(* Logix 5000 AddOnInstructionDefinition export Banner_K50Select_Param_v4; software revision 33.03 *)

TYPE Banner_IOL_Port_v4 :   // UDT that has all of the data items necessary to communicate with a specific Port on a IO-Link Master
STRUCT
   Port_Controlled : INT;   // Each bit represents a port on an IO-Link Master. Set to 1 to tell AOI to control that port.
   Port_Activate : INT;   // Each bit represents a port on an IO-Link Master. When ON that port will process any commands in queue.
   Port_Read : INT;   // Each bit represents a port on an IO-Link Master. Used to determine when device AOI has requested a Read command.
   Port_Write : INT;   // Each bit represents a port on an IO-Link Master. Used to determine when device AOI has requested a Write command.
   Port_RW_Complete : INT;   // Each bit represents a port on an IO-Link Master. Tells device AOI that Read or Write request has been completed.
   Port_Device_Read : INT;
   Data_Transfer : SINT[190];   // Array to transfer data from IO-Master to device AOIs.
END_STRUCT
END_TYPE

TYPE Banner_K50Select_DeviceLocks_v4 :
STRUCT
   Parameter_Access_Lock : SINT;   // Write access to all read/write parameters is block when this bit is ON.
   Data_Storage_Lock : SINT;   // Data storage mechanism is inhibited when bit is ON.
   Local_Parameterization_Lock : SINT;   // Parameteriation via local control elementes is inhibited.
   Local_User_Interface_Lock : SINT;   // Operation of the hmi on the device is disabled.
END_STRUCT
END_TYPE

TYPE Banner_K50Select_Direct_v4 :
STRUCT
   Master_Cycle_Time : INT;
   Min_Cycle_Time : INT;
   M_Sequence_Capability : INT;
   IO_Link_Version_ID : INT;
   Process_Data_Input_Length : INT;
   Process_Data_Output_Length : INT;
   Combined_Vendor_ID : DINT;   // IO-Link Vendor ID
   Vendor_ID1 : INT;
   Vendor_ID2 : INT;
   Combined_Device_ID : DINT;   // IO-Link Device ID
   Device_ID1 : INT;
   Device_ID2 : INT;
   Device_ID3 : INT;
END_STRUCT
END_TYPE

TYPE Banner_K50Select_InputSettings_v4 :
STRUCT
   Touch_Sensitivity : SINT;   // K50 Select touch models only. 0 = Low, 1 = High.
   Function : SINT;   // 0 = Momentary, 1 = Latched.
   Mute_Enable : SINT;   // 0 = Off, 1 = On.
   On_Delay : DINT;   // 0 to 65535 in ms. Length of time the touch button needs to be pressed to trigger touch active state.
   Target_Threshold_Low : DINT;   // K50 Select Sensor Models Only. 0 to 1500 Range in mm.
   Targer_Threshold_High : DINT;   // K50 Select Sensor Models Only. 0 to 1500 Range in mm.
   Min_Distance : DINT;   // K50 Select Sensor Models Only. 0 to 1500 Range in mm.
   Max_Distance : DINT;   // K50 Select Sensor Models Only. 0 to 1500 Range in mm.
END_STRUCT
END_TYPE

TYPE Banner_K50Select_Output_Settings_v4 :
STRUCT
   Output_State : SINT;   // 0 = NO, 1 = NC.
   Off_Delay_Type : SINT;   // 0 = Leading Edge, 1 = Trailing Edge.
   Off_Delay : DINT;   // 0 to 65535 in ms. Length of time before the device returns to the 'touch inactive' state after button is released.
END_STRUCT
END_TYPE

TYPE Banner_K50Select_RD_v4 :   // UDT with all of the Read only parameters for K50 Pro Select.
STRUCT
   Direct_Parameters : Banner_K50Select_Direct_v4;
   Serial_Number : STRING;
END_STRUCT
END_TYPE

TYPE Banner_K50Select_Settings_v4 :
STRUCT
   Custom_Intensity : SINT;   // 0 to 100 %
   Custom_Flash_Rate : INT;   // Range 5 to 200 (.5 to 20 converted rate).
   Restrict_to_Gamut : SINT;   // 0 = Off, 1 = On.
END_STRUCT
END_TYPE

TYPE Banner_K50Select_SP_v4 :   // UDT for K50 Pro Select with the State Parameters structure.
STRUCT
   Animation_Type : SINT;   // 0 = Off, 1 = Steady, 2 = Flash, 3 = Two Color Flash, 4 = 50/50, 5 = 50/50 Rotate, 6 = Chase, 7 = Intensity Sweep, 8 = Sequence.
   Direction : SINT;   // 0 = CCW, 1 = CW.
   Pattern : SINT;   // 0 = Flash, 1 = Strobe, 2 = Three Pulse, 3 = SOS, 4 = Random.
   Speed : SINT;   // 0 = Slow, 1 = Medium, 2 = Fast, 3 = Custom.
   Reserved : SINT;
   Off_Delay_Type : SINT;   // 0 =Leading Edge, 1 = Trailing Edge.
   Off_Delay : DINT;   // 0 to 65535 in ms. Length of time before the device returns to 'touch inactive' state after button is released.
   Static_Sequence : INT;   // 0 to 255. Value describing the LED position of the device.
   Sequence_Start_Location : SINT;   // 0 = LED1, 1 = LED2, 2 = LED3, 3 = LED4, 4 = LED5, 5 = LED6, 6 = LED7, 7 = LED8.
   Color_1 : SINT;   // 0 = Green, 1 = Red, 2 = Orange, 3 = Amber, 4 = Yellow, 5 = Lime Green, 6 = Spring Green, 7 = Cyan, 8 = SKy Blue, 9 = Blue, 10 = Violet, 11 = Magenta, 12 = Rose, 13 = White, 14 Custom 1, 15 = Custom 2.
   Color_1_Intensity : SINT;   // 0 = High, 1 = Medium, 2 = Low, 3 = Off, 4 = Custom.
   Color_2 : SINT;   // 0 = Green, 1 = Red, 2 = Orange, 3 = Amber, 4 = Yellow, 5 = Lime Green, 6 = Spring Green, 7 = Cyan, 8 = SKy Blue, 9 = Blue, 10 = Violet, 11 = Magenta, 12 = Rose, 13 = White, 14 Custom 1, 15 = Custom 2.
   Color_2_Intensity : SINT;   // 0 = High, 1 = Medium, 2 = Low, 3 = Off, 4 = Custom.
   Min_Distance : DINT;   // Only for K50 Pro Select Sensor Model. 0 to 1500 mm.
   Max_Distance : DINT;   // Only for K50 Pro Select Sensor Model. 0 to 1500 mm.
   Output_State : SINT;   // Only for K50 Pro Select Sensor Model. 0=False, 1=True.
END_STRUCT
END_TYPE

TYPE Banner_K50Select_v4 :   // UDT with all of the parameters for K50 Pro Select.
STRUCT
   Initial_Global_Read : BOOL;   // Determines if all of the IO-Link data has been read into the PLC yet
   Command : INT;   // Value placed in here will activate a read or write to a specifc IO-Link Index
   Read : Banner_K50Select_RD_v4;   // All read data
   Write : Banner_K50Select_WD_v4;   // All data that can be written to.
   Archive : Banner_K50Select_WD_v4;   // Archive of the write data.
   Reset : BOOL;
END_STRUCT
END_TYPE

TYPE Banner_K50Select_WD_v4 :   // UDT that stores the Write Data for a K50 Pro Select.
STRUCT
   System_Command : INT;   // See IODD file for list of commands that can be activated via the System Command interface
   Device_Access_Locks : Banner_K50Select_DeviceLocks_v4;
   Operation_Mode : SINT;   // 0 = Multicolor, 1 = Four State Full Logic, 2 = Advanced, 3 = LED Control, 4 = Demo.
   Settings : Banner_K50Select_Settings_v4;
   Input_Settings : Banner_K50Select_InputSettings_v4;
   Output_Settings : Banner_K50Select_Output_Settings_v4;
   State_Parameters : Banner_K50Select_SP_v4[6];   // State Parameters. 1 through 4 will have values.
   CC1_Red : INT;   // 0-255. Custom 1 Red.
   CC1_Green : INT;   // 0-255. Custom 1 Green.
   CC1_Blue : INT;   // 0-255. Custom 1 Blue.
   CC2_Red : INT;   // 0-255. Custom 2 Red.
   CC2_Green : INT;   // 0-255. Custom 2 Green.
   CC2_Blue : INT;   // 0-255. Custom 2 Blue.
END_STRUCT
END_TYPE

ADD_ON_INSTRUCTION Banner_K50Select_Param_v4   (* revision 4.2, vendor Banner Engineering *)
// AOI to read and write parameter data to an IO-Link K50 Pro Select.
VAR_IN_OUT
   K50 : Banner_K50Select_v4; {required}
   Port_Data : Banner_IOL_Port_v4; {required}
END_VAR
VAR_INPUT
   Port : DINT; {required}
   Type : DINT; {required}   // 1=Sensor, 2=Touch, 3=Indicator
END_VAR
VAR
   Local_Control : DINT; {access None}
   Global_Read_Command_Value : INT; {access None}
   Global_Write_Command_Value : INT; {access None}
   Command_Being_Processed : BOOL; {access None}
   Update_Archive : BOOL; {access None}
   Index_Write_Control : DINT; {access None}
   Index_Write_Inprocess : INT; {access None}
   Temp_Excess_Gain : DINT[2]; {access None}
   Inprocess_Index : DINT; {access None}
   SP_Index : DINT; {access None}   // State Parameters Index
   SP_Write_Index : DINT; {access None}
   SP_R_Index : DINT; {access None}
   SP_W_Index : DINT; {access None}
END_VAR

ROUTINE Logic   (* ladder *)
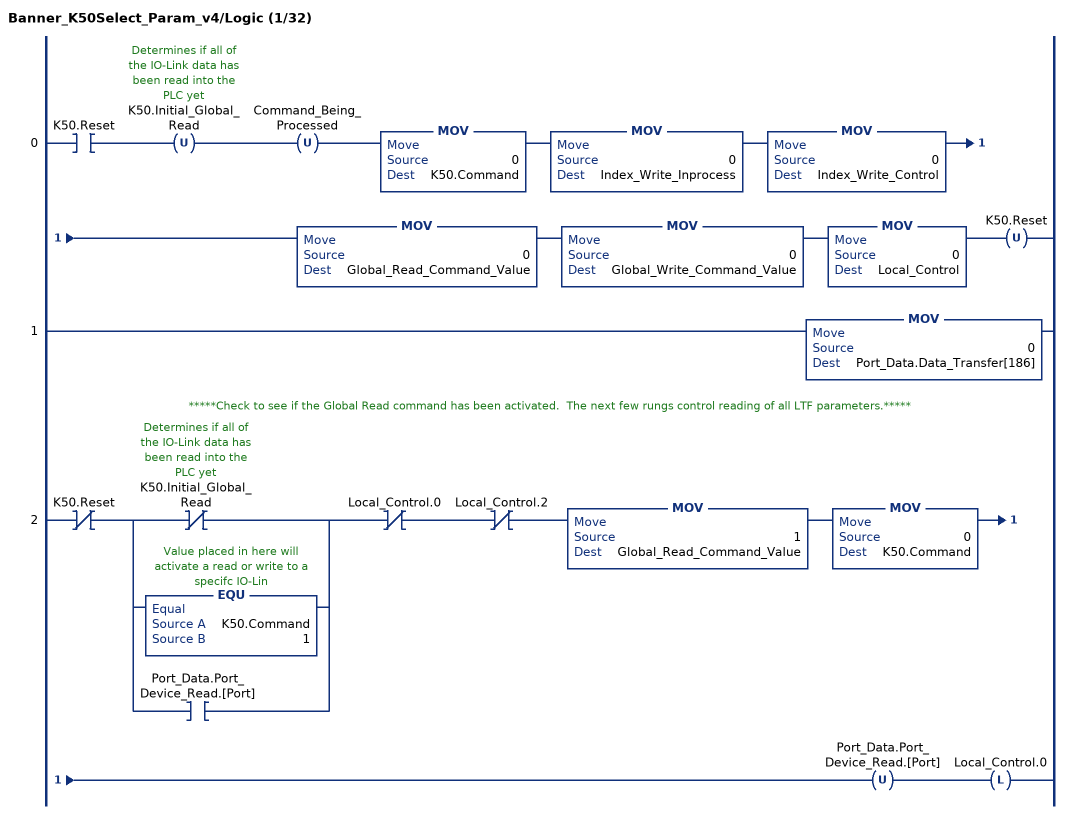
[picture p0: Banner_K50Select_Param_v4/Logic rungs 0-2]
   0: XIC(K50.Reset)OTU(K50.Initial_Global_Read)OTU(Command_Being_Processed)MOV(0,K50.Command)MOV(0,Index_Write_Inprocess)MOV(0,Index_Write_Control)MOV(0,Global_Read_Command_Value)MOV(0,Global_Write_Command_Value)MOV(0,Local_Control)OTU(K50.Reset);
   1: MOV(0,Port_Data.Data_Transfer[186]);
   // *****Check to see if the Global Read command has been activated.  The next few rungs control reading of all LTF parameters.*****
   2: XIO(K50.Reset)[XIO(K50.Initial_Global_Read) ,EQU(K50.Command,1) ,XIC(Port_Data.Port_Device_Read.[Port]) ]XIO(Local_Control.0)XIO(Local_Control.2)MOV(1,Global_Read_Command_Value)MOV(0,K50.Command)OTU(Port_Data.Port_Device_Read.[Port])OTL(Local_Control.0);
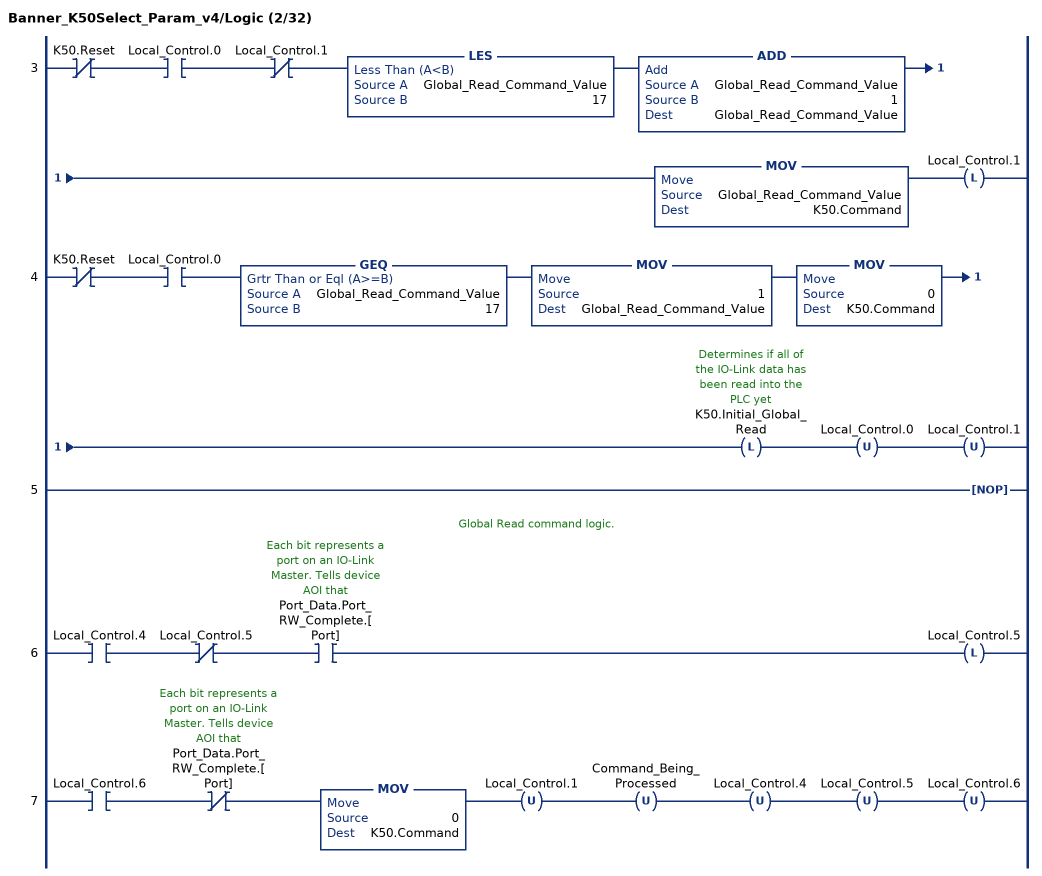
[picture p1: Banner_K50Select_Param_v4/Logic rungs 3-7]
   3: XIO(K50.Reset)XIC(Local_Control.0)XIO(Local_Control.1)LES(Global_Read_Command_Value,17)ADD(Global_Read_Command_Value,1,Global_Read_Command_Value)MOV(Global_Read_Command_Value,K50.Command)OTL(Local_Control.1);
   4: XIO(K50.Reset)XIC(Local_Control.0)GEQ(Global_Read_Command_Value,17)MOV(1,Global_Read_Command_Value)MOV(0,K50.Command)OTL(K50.Initial_Global_Read)OTU(Local_Control.0)OTU(Local_Control.1);
   5: NOP();
   // Global Read command logic.
   6: XIC(Local_Control.4)XIO(Local_Control.5)XIC(Port_Data.Port_RW_Complete.[Port])OTL(Local_Control.5);
   7: XIC(Local_Control.6)XIO(Port_Data.Port_RW_Complete.[Port])MOV(0,K50.Command)OTU(Local_Control.1)OTU(Command_Being_Processed)OTU(Local_Control.4)OTU(Local_Control.5)OTU(Local_Control.6);
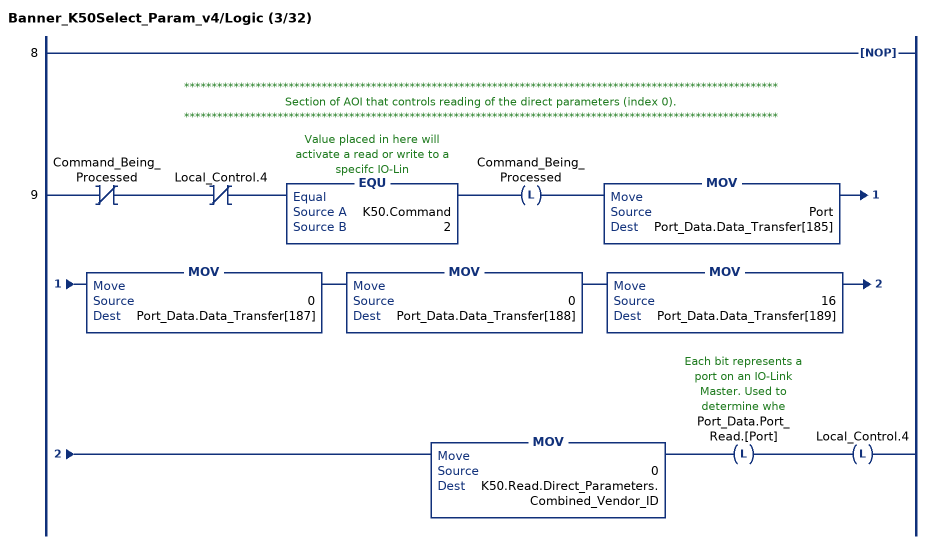
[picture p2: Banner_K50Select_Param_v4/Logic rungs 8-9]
   8: NOP();
   // ************************************************************************************************************
   // Section of AOI that controls reading of the direct parameters (index 0).
   // ************************************************************************************************************
   9: XIO(Command_Being_Processed)XIO(Local_Control.4)EQU(K50.Command,2)OTL(Command_Being_Processed)MOV(Port,Port_Data.Data_Transfer[185])MOV(0,Port_Data.Data_Transfer[187])MOV(0,Port_Data.Data_Transfer[188])MOV(16,Port_Data.Data_Transfer[189])MOV(0,K50.Read.Direct_Parameters.Combined_Vendor_ID)OTL(Port_Data.Port_Read.[Port])OTL(Local_Control.4);
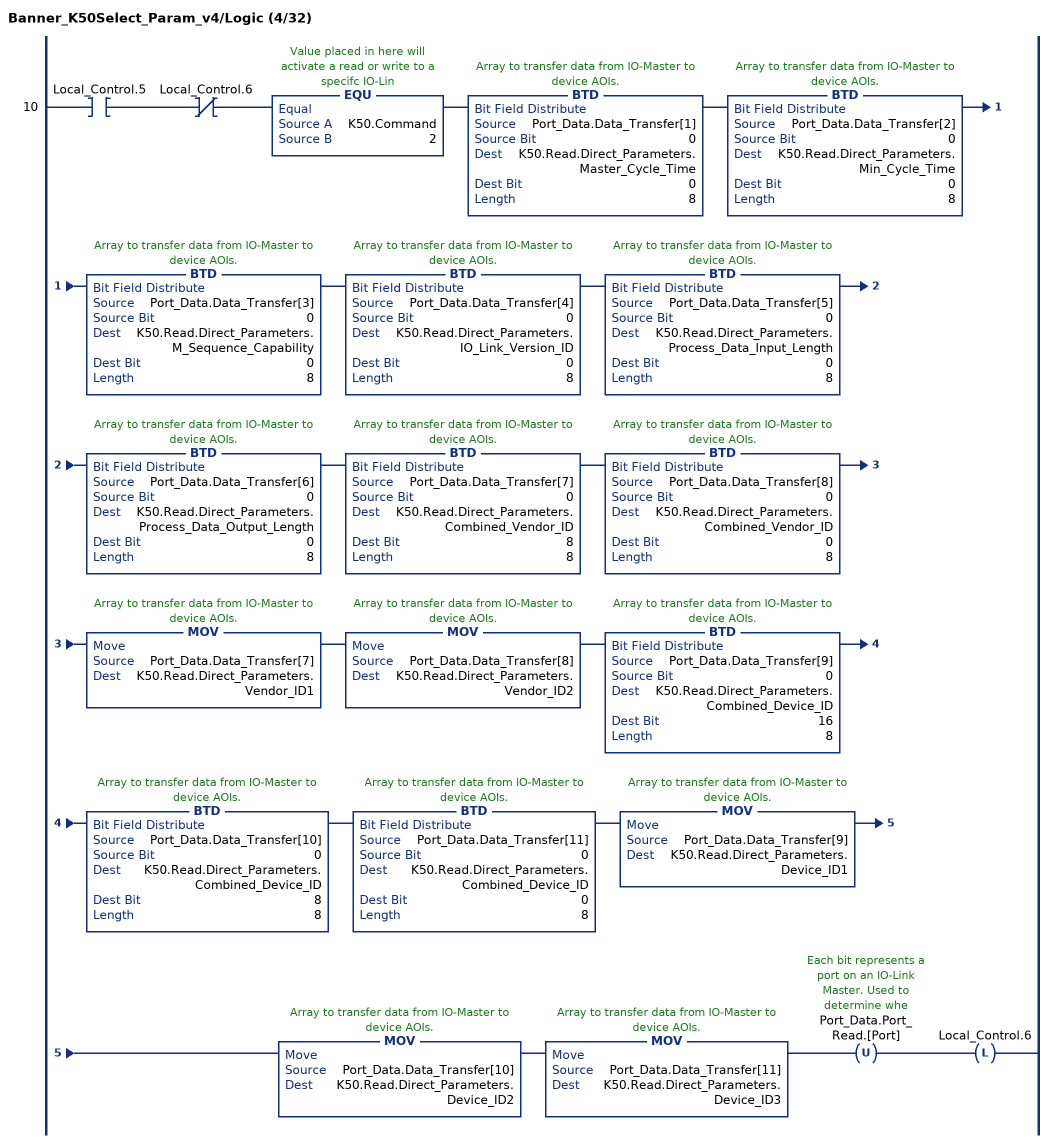
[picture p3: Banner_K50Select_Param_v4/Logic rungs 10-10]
   10: XIC(Local_Control.5)XIO(Local_Control.6)EQU(K50.Command,2)BTD(Port_Data.Data_Transfer[1],0,K50.Read.Direct_Parameters.Master_Cycle_Time,0,8)BTD(Port_Data.Data_Transfer[2],0,K50.Read.Direct_Parameters.Min_Cycle_Time,0,8)BTD(Port_Data.Data_Transfer[3],0,K50.Read.Direct_Parameters.M_Sequence_Capability,0,8)BTD(Port_Data.Data_Transfer[4],0,K50.Read.Direct_Parameters.IO_Link_Version_ID,0,8)BTD(Port_Data.Data_Transfer[5],0,K50.Read.Direct_Parameters.Process_Data_Input_Length,0,8)BTD(Port_Data.Data_Transfer[6],0,K50.Read.Direct_Parameters.Process_Data_Output_Length,0,8)BTD(Port_Data.Data_Transfer[7],0,K50.Read.Direct_Parameters.Combined_Vendor_ID,8,8)BTD(Port_Data.Data_Transfer[8],0,K50.Read.Direct_Parameters.Combined_Vendor_ID,0,8)MOV(Port_Data.Data_Transfer[7],K50.Read.Direct_Parameters.Vendor_ID1)MOV(Port_Data.Data_Transfer[8],K50.Read.Direct_Parameters.Vendor_ID2)BTD(Port_Data.Data_Transfer[9],0,K50.Read.Direct_Parameters.Combined_Device_ID,16,8)BTD(Port_Data.Data_Transfer[10],0,K50.Read.Direct_Parameters.Combined_Device_ID,8,8)BTD(Port_Data.Data_Transfer[11],0,K50.Read.Direct_Parameters.Combined_Device_ID,0,8)MOV(Port_Data.Data_Transfer[9],K50.Read.Direct_Parameters.Device_ID1)MOV(Port_Data.Data_Transfer[10],K50.Read.Direct_Parameters.Device_ID2)MOV(Port_Data.Data_Transfer[11],K50.Read.Direct_Parameters.Device_ID3)OTU(Port_Data.Port_Read.[Port])OTL(Local_Control.6);
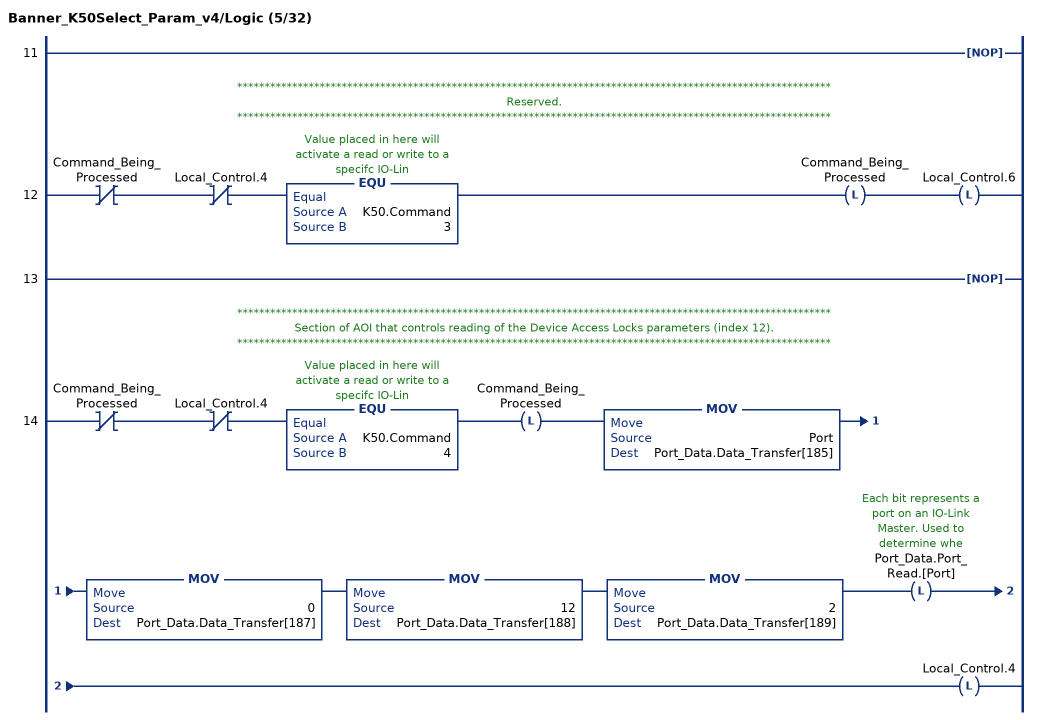
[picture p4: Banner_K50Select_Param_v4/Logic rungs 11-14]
   11: NOP();
   // ************************************************************************************************************
   // Reserved.
   // ************************************************************************************************************
   12: XIO(Command_Being_Processed)XIO(Local_Control.4)EQU(K50.Command,3)OTL(Command_Being_Processed)OTL(Local_Control.6);
   13: NOP();
   // ************************************************************************************************************
   // Section of AOI that controls reading of the Device Access Locks parameters (index 12).
   // ************************************************************************************************************
   14: XIO(Command_Being_Processed)XIO(Local_Control.4)EQU(K50.Command,4)OTL(Command_Being_Processed)MOV(Port,Port_Data.Data_Transfer[185])MOV(0,Port_Data.Data_Transfer[187])MOV(12,Port_Data.Data_Transfer[188])MOV(2,Port_Data.Data_Transfer[189])OTL(Port_Data.Port_Read.[Port])OTL(Local_Control.4);
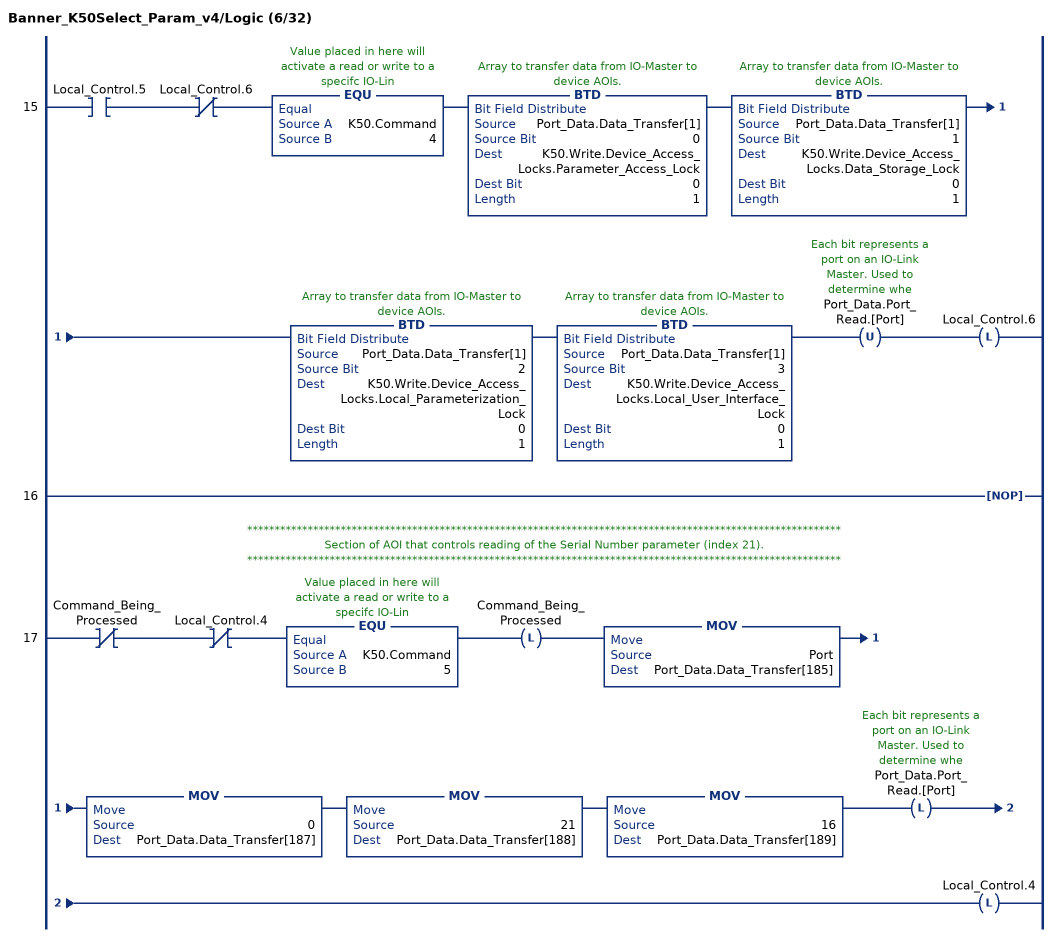
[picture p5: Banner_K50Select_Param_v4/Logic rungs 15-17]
   15: XIC(Local_Control.5)XIO(Local_Control.6)EQU(K50.Command,4)BTD(Port_Data.Data_Transfer[1],0,K50.Write.Device_Access_Locks.Parameter_Access_Lock,0,1)BTD(Port_Data.Data_Transfer[1],1,K50.Write.Device_Access_Locks.Data_Storage_Lock,0,1)BTD(Port_Data.Data_Transfer[1],2,K50.Write.Device_Access_Locks.Local_Parameterization_Lock,0,1)BTD(Port_Data.Data_Transfer[1],3,K50.Write.Device_Access_Locks.Local_User_Interface_Lock,0,1)OTU(Port_Data.Port_Read.[Port])OTL(Local_Control.6);
   16: NOP();
   // ************************************************************************************************************
   // Section of AOI that controls reading of the Serial Number parameter (index 21).
   // ************************************************************************************************************
   17: XIO(Command_Being_Processed)XIO(Local_Control.4)EQU(K50.Command,5)OTL(Command_Being_Processed)MOV(Port,Port_Data.Data_Transfer[185])MOV(0,Port_Data.Data_Transfer[187])MOV(21,Port_Data.Data_Transfer[188])MOV(16,Port_Data.Data_Transfer[189])OTL(Port_Data.Port_Read.[Port])OTL(Local_Control.4);
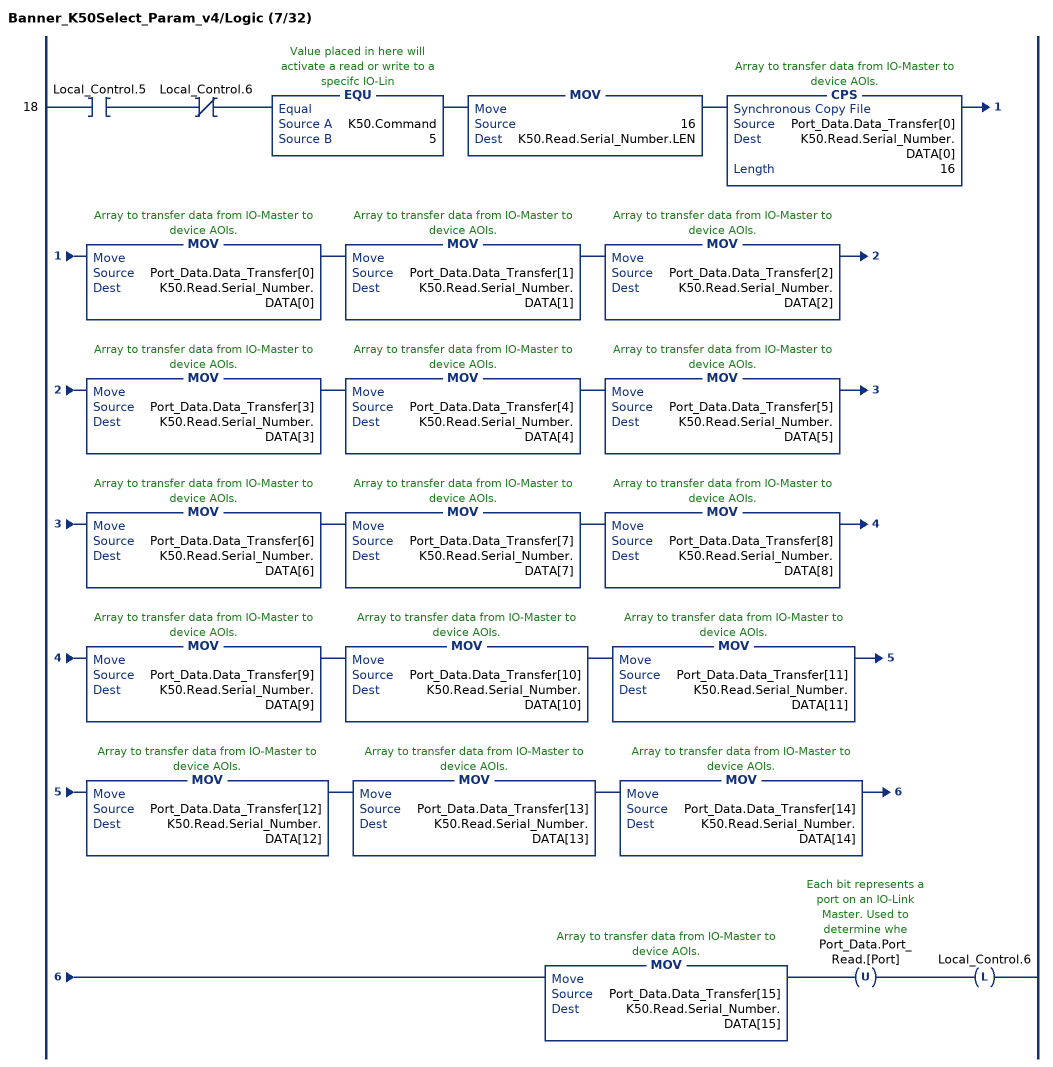
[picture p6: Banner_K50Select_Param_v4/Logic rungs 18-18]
   18: XIC(Local_Control.5)XIO(Local_Control.6)EQU(K50.Command,5)MOV(16,K50.Read.Serial_Number.LEN)CPS(Port_Data.Data_Transfer[0],K50.Read.Serial_Number.DATA[0],16)MOV(Port_Data.Data_Transfer[0],K50.Read.Serial_Number.DATA[0])MOV(Port_Data.Data_Transfer[1],K50.Read.Serial_Number.DATA[1])MOV(Port_Data.Data_Transfer[2],K50.Read.Serial_Number.DATA[2])MOV(Port_Data.Data_Transfer[3],K50.Read.Serial_Number.DATA[3])MOV(Port_Data.Data_Transfer[4],K50.Read.Serial_Number.DATA[4])MOV(Port_Data.Data_Transfer[5],K50.Read.Serial_Number.DATA[5])MOV(Port_Data.Data_Transfer[6],K50.Read.Serial_Number.DATA[6])MOV(Port_Data.Data_Transfer[7],K50.Read.Serial_Number.DATA[7])MOV(Port_Data.Data_Transfer[8],K50.Read.Serial_Number.DATA[8])MOV(Port_Data.Data_Transfer[9],K50.Read.Serial_Number.DATA[9])MOV(Port_Data.Data_Transfer[10],K50.Read.Serial_Number.DATA[10])MOV(Port_Data.Data_Transfer[11],K50.Read.Serial_Number.DATA[11])MOV(Port_Data.Data_Transfer[12],K50.Read.Serial_Number.DATA[12])MOV(Port_Data.Data_Transfer[13],K50.Read.Serial_Number.DATA[13])MOV(Port_Data.Data_Transfer[14],K50.Read.Serial_Number.DATA[14])MOV(Port_Data.Data_Transfer[15],K50.Read.Serial_Number.DATA[15])OTU(Port_Data.Port_Read.[Port])OTL(Local_Control.6);
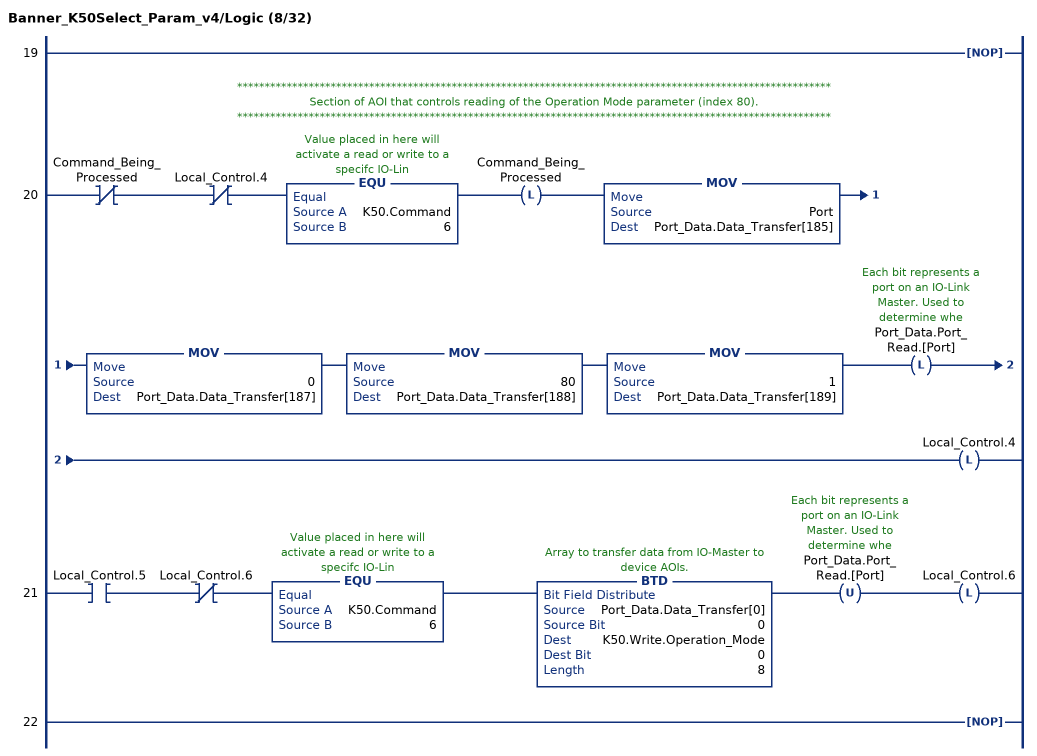
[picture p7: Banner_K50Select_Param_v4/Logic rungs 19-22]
   19: NOP();
   // ************************************************************************************************************
   // Section of AOI that controls reading of the Operation Mode parameter (index 80).
   // ************************************************************************************************************
   20: XIO(Command_Being_Processed)XIO(Local_Control.4)EQU(K50.Command,6)OTL(Command_Being_Processed)MOV(Port,Port_Data.Data_Transfer[185])MOV(0,Port_Data.Data_Transfer[187])MOV(80,Port_Data.Data_Transfer[188])MOV(1,Port_Data.Data_Transfer[189])OTL(Port_Data.Port_Read.[Port])OTL(Local_Control.4);
   21: XIC(Local_Control.5)XIO(Local_Control.6)EQU(K50.Command,6)BTD(Port_Data.Data_Transfer[0],0,K50.Write.Operation_Mode,0,8)OTU(Port_Data.Port_Read.[Port])OTL(Local_Control.6);
   22: NOP();
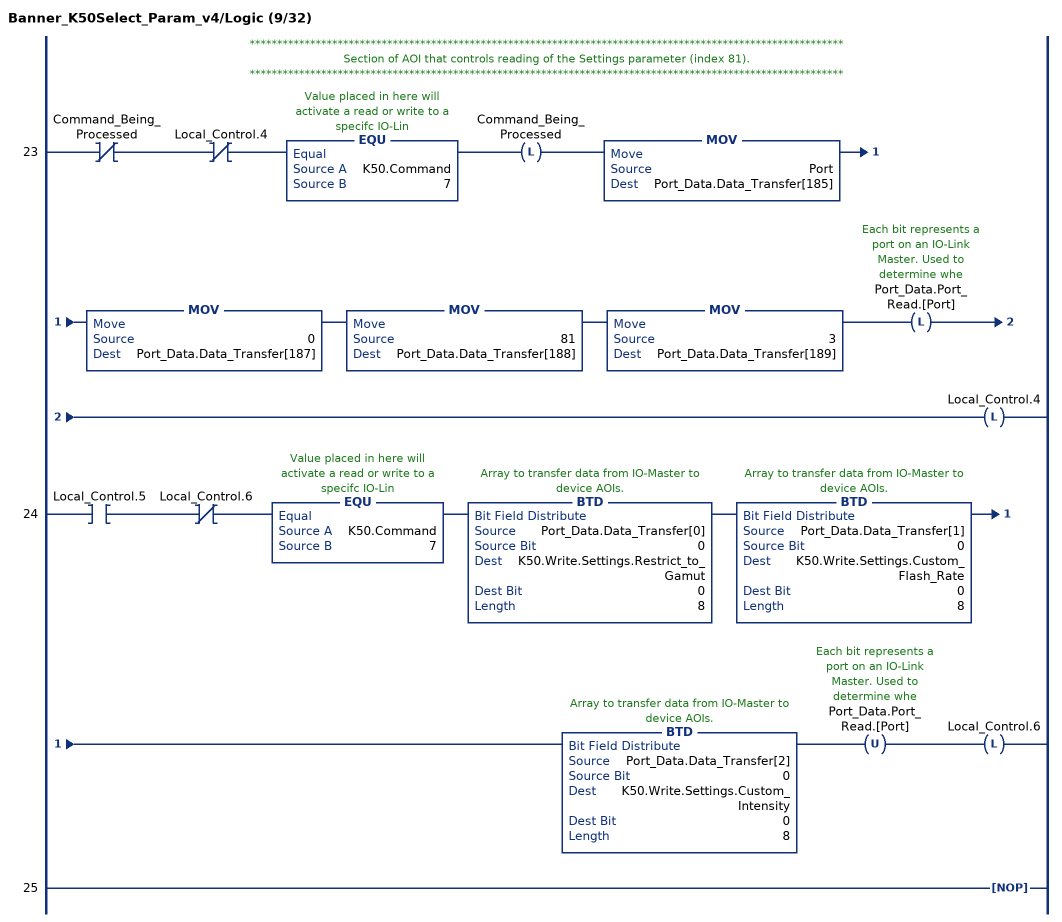
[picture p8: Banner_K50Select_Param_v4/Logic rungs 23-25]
   // ************************************************************************************************************
   // Section of AOI that controls reading of the Settings parameter (index 81).
   // ************************************************************************************************************
   23: XIO(Command_Being_Processed)XIO(Local_Control.4)EQU(K50.Command,7)OTL(Command_Being_Processed)MOV(Port,Port_Data.Data_Transfer[185])MOV(0,Port_Data.Data_Transfer[187])MOV(81,Port_Data.Data_Transfer[188])MOV(3,Port_Data.Data_Transfer[189])OTL(Port_Data.Port_Read.[Port])OTL(Local_Control.4);
   24: XIC(Local_Control.5)XIO(Local_Control.6)EQU(K50.Command,7)BTD(Port_Data.Data_Transfer[0],0,K50.Write.Settings.Restrict_to_Gamut,0,8)BTD(Port_Data.Data_Transfer[1],0,K50.Write.Settings.Custom_Flash_Rate,0,8)BTD(Port_Data.Data_Transfer[2],0,K50.Write.Settings.Custom_Intensity,0,8)OTU(Port_Data.Port_Read.[Port])OTL(Local_Control.6);
   25: NOP();
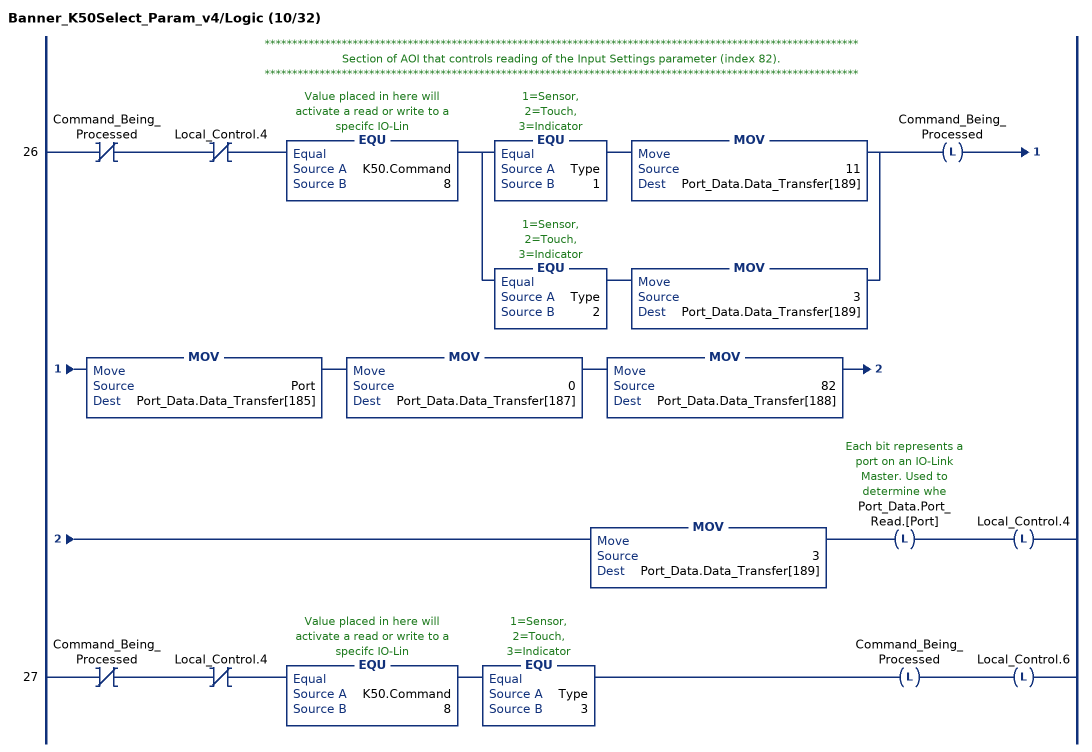
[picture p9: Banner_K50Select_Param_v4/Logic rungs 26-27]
   // ************************************************************************************************************
   // Section of AOI that controls reading of the Input Settings parameter (index 82).
   // ************************************************************************************************************
   26: XIO(Command_Being_Processed)XIO(Local_Control.4)EQU(K50.Command,8)[EQU(Type,1) MOV(11,Port_Data.Data_Transfer[189]) ,EQU(Type,2) MOV(3,Port_Data.Data_Transfer[189]) ]OTL(Command_Being_Processed)MOV(Port,Port_Data.Data_Transfer[185])MOV(0,Port_Data.Data_Transfer[187])MOV(82,Port_Data.Data_Transfer[188])MOV(3,Port_Data.Data_Transfer[189])OTL(Port_Data.Port_Read.[Port])OTL(Local_Control.4);
   27: XIO(Command_Being_Processed)XIO(Local_Control.4)EQU(K50.Command,8)EQU(Type,3)OTL(Command_Being_Processed)OTL(Local_Control.6);
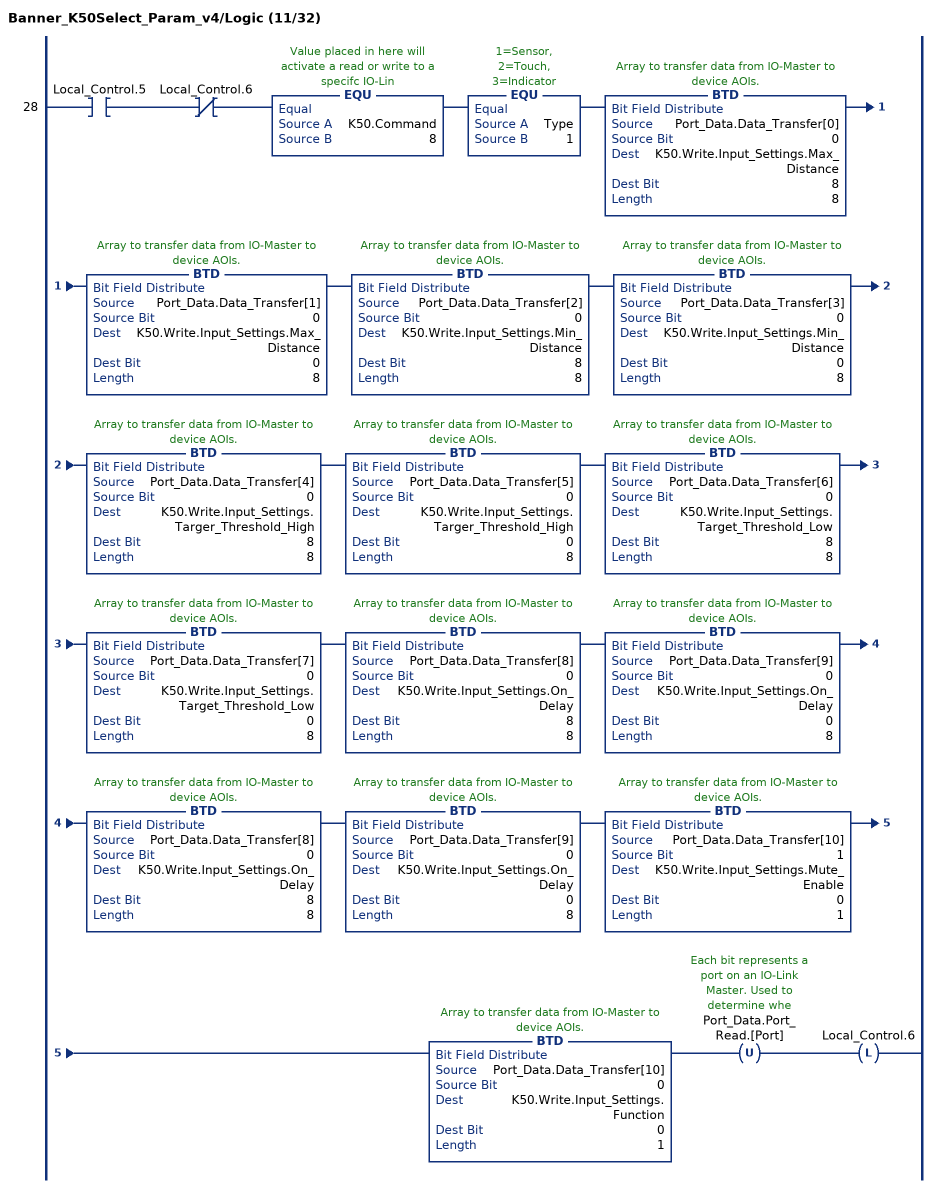
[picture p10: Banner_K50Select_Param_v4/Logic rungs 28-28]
   28: XIC(Local_Control.5)XIO(Local_Control.6)EQU(K50.Command,8)EQU(Type,1)BTD(Port_Data.Data_Transfer[0],0,K50.Write.Input_Settings.Max_Distance,8,8)BTD(Port_Data.Data_Transfer[1],0,K50.Write.Input_Settings.Max_Distance,0,8)BTD(Port_Data.Data_Transfer[2],0,K50.Write.Input_Settings.Min_Distance,8,8)BTD(Port_Data.Data_Transfer[3],0,K50.Write.Input_Settings.Min_Distance,0,8)BTD(Port_Data.Data_Transfer[4],0,K50.Write.Input_Settings.Targer_Threshold_High,8,8)BTD(Port_Data.Data_Transfer[5],0,K50.Write.Input_Settings.Targer_Threshold_High,0,8)BTD(Port_Data.Data_Transfer[6],0,K50.Write.Input_Settings.Target_Threshold_Low,8,8)BTD(Port_Data.Data_Transfer[7],0,K50.Write.Input_Settings.Target_Threshold_Low,0,8)BTD(Port_Data.Data_Transfer[8],0,K50.Write.Input_Settings.On_Delay,8,8)BTD(Port_Data.Data_Transfer[9],0,K50.Write.Input_Settings.On_Delay,0,8)BTD(Port_Data.Data_Transfer[8],0,K50.Write.Input_Settings.On_Delay,8,8)BTD(Port_Data.Data_Transfer[9],0,K50.Write.Input_Settings.On_Delay,0,8)BTD(Port_Data.Data_Transfer[10],1,K50.Write.Input_Settings.Mute_Enable,0,1)BTD(Port_Data.Data_Transfer[10],0,K50.Write.Input_Settings.Function,0,1)OTU(Port_Data.Port_Read.[Port])OTL(Local_Control.6);
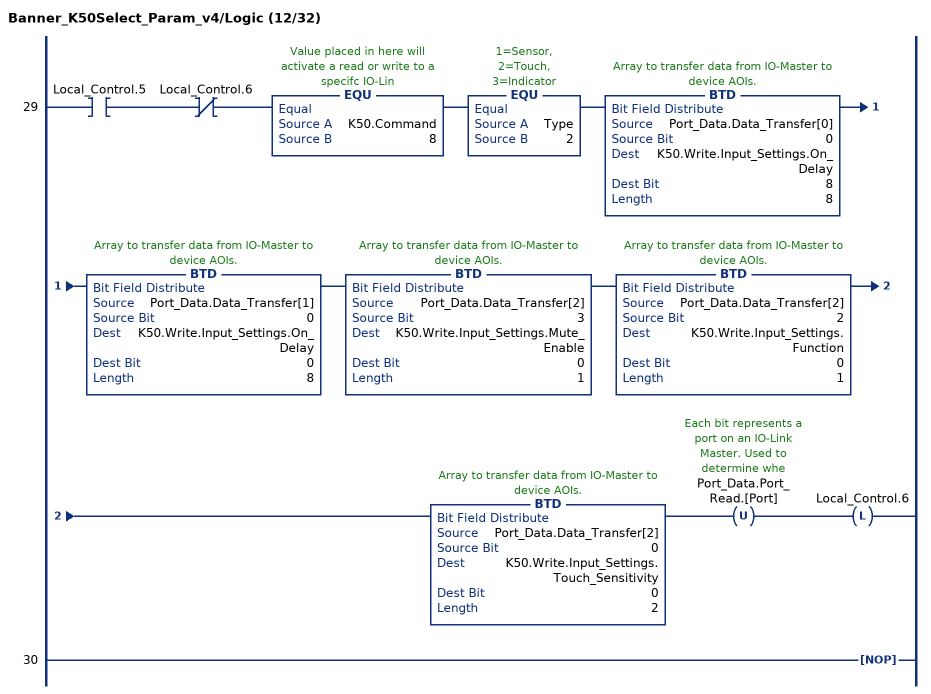
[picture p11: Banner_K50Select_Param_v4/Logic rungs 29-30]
   29: XIC(Local_Control.5)XIO(Local_Control.6)EQU(K50.Command,8)EQU(Type,2)BTD(Port_Data.Data_Transfer[0],0,K50.Write.Input_Settings.On_Delay,8,8)BTD(Port_Data.Data_Transfer[1],0,K50.Write.Input_Settings.On_Delay,0,8)BTD(Port_Data.Data_Transfer[2],3,K50.Write.Input_Settings.Mute_Enable,0,1)BTD(Port_Data.Data_Transfer[2],2,K50.Write.Input_Settings.Function,0,1)BTD(Port_Data.Data_Transfer[2],0,K50.Write.Input_Settings.Touch_Sensitivity,0,2)OTU(Port_Data.Port_Read.[Port])OTL(Local_Control.6);
   30: NOP();
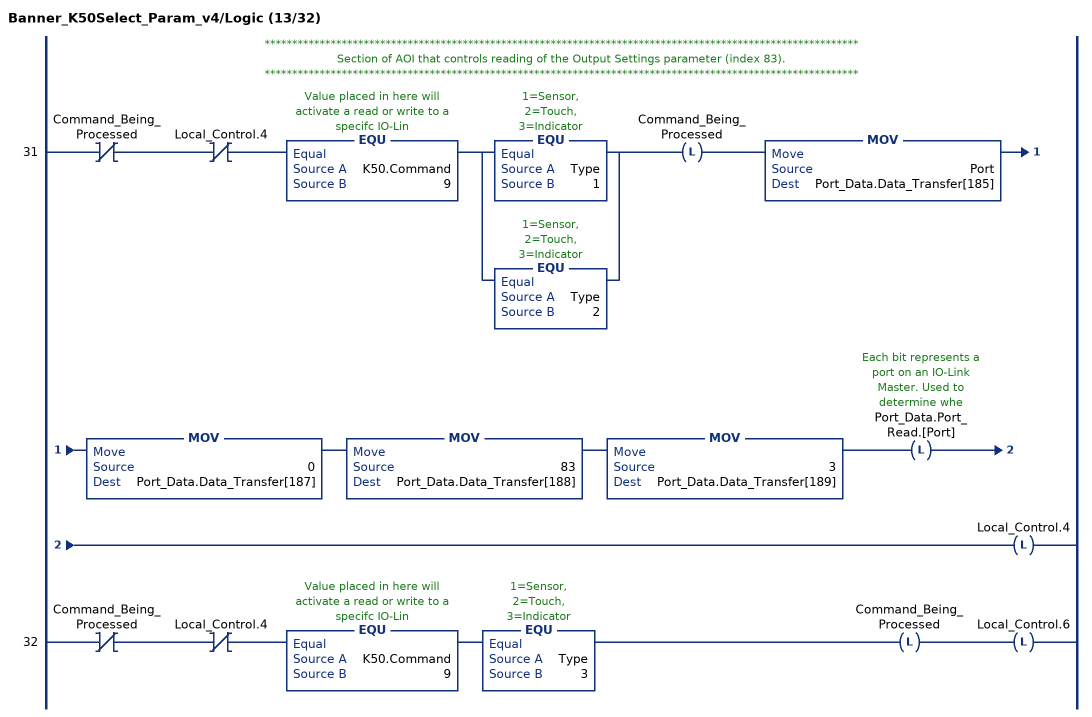
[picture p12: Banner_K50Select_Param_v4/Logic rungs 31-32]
   // ************************************************************************************************************
   // Section of AOI that controls reading of the Output Settings parameter (index 83).
   // ************************************************************************************************************
   31: XIO(Command_Being_Processed)XIO(Local_Control.4)EQU(K50.Command,9)[EQU(Type,1) ,EQU(Type,2) ]OTL(Command_Being_Processed)MOV(Port,Port_Data.Data_Transfer[185])MOV(0,Port_Data.Data_Transfer[187])MOV(83,Port_Data.Data_Transfer[188])MOV(3,Port_Data.Data_Transfer[189])OTL(Port_Data.Port_Read.[Port])OTL(Local_Control.4);
   32: XIO(Command_Being_Processed)XIO(Local_Control.4)EQU(K50.Command,9)EQU(Type,3)OTL(Command_Being_Processed)OTL(Local_Control.6);
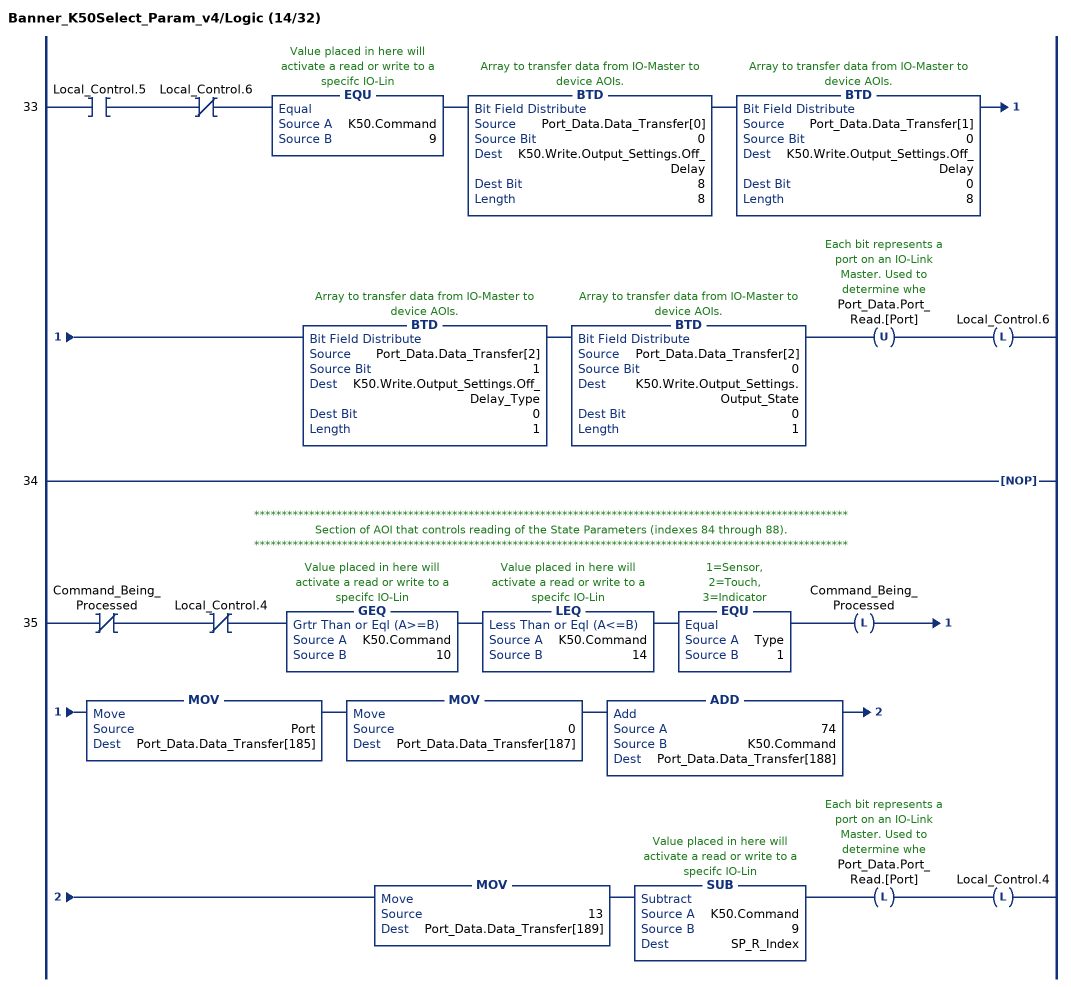
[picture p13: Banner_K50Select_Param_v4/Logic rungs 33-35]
   33: XIC(Local_Control.5)XIO(Local_Control.6)EQU(K50.Command,9)BTD(Port_Data.Data_Transfer[0],0,K50.Write.Output_Settings.Off_Delay,8,8)BTD(Port_Data.Data_Transfer[1],0,K50.Write.Output_Settings.Off_Delay,0,8)BTD(Port_Data.Data_Transfer[2],1,K50.Write.Output_Settings.Off_Delay_Type,0,1)BTD(Port_Data.Data_Transfer[2],0,K50.Write.Output_Settings.Output_State,0,1)OTU(Port_Data.Port_Read.[Port])OTL(Local_Control.6);
   34: NOP();
   // ************************************************************************************************************
   // Section of AOI that controls reading of the State Parameters (indexes 84 through 88).
   // ************************************************************************************************************
   35: XIO(Command_Being_Processed)XIO(Local_Control.4)GEQ(K50.Command,10)LEQ(K50.Command,14)EQU(Type,1)OTL(Command_Being_Processed)MOV(Port,Port_Data.Data_Transfer[185])MOV(0,Port_Data.Data_Transfer[187])ADD(74,K50.Command,Port_Data.Data_Transfer[188])MOV(13,Port_Data.Data_Transfer[189])SUB(K50.Command,9,SP_R_Index)OTL(Port_Data.Port_Read.[Port])OTL(Local_Control.4);
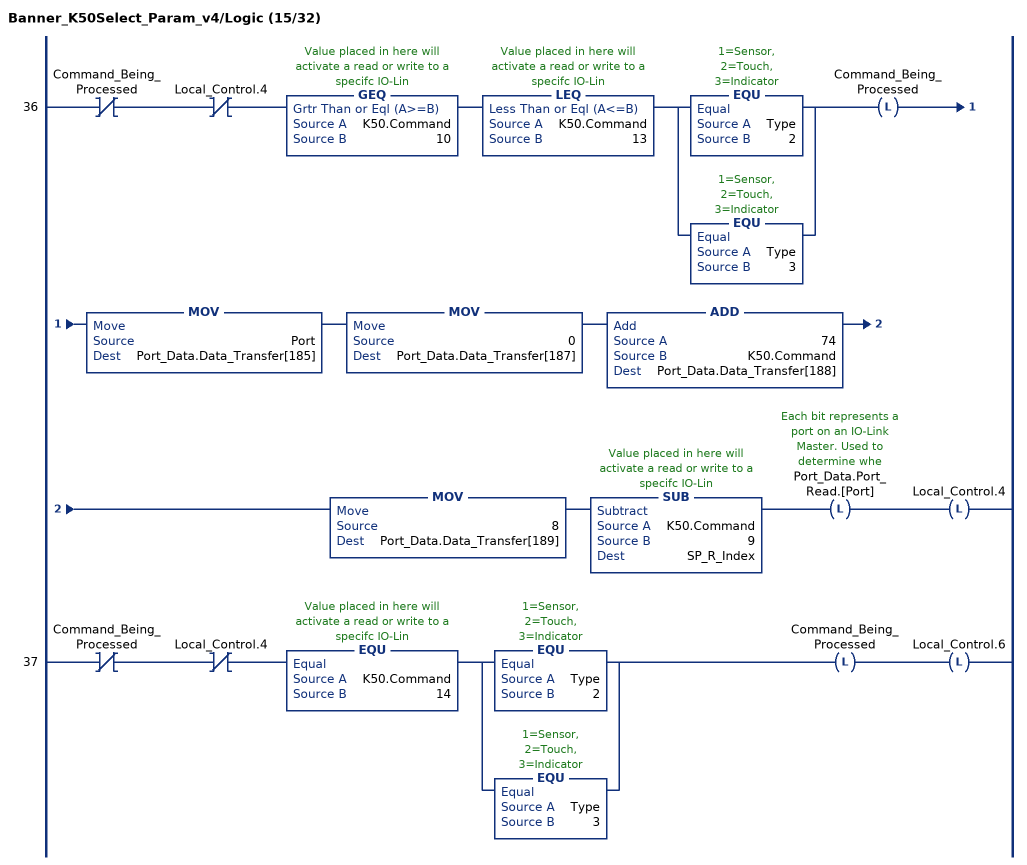
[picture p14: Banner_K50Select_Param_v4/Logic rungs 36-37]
   36: XIO(Command_Being_Processed)XIO(Local_Control.4)GEQ(K50.Command,10)LEQ(K50.Command,13)[EQU(Type,2) ,EQU(Type,3) ]OTL(Command_Being_Processed)MOV(Port,Port_Data.Data_Transfer[185])MOV(0,Port_Data.Data_Transfer[187])ADD(74,K50.Command,Port_Data.Data_Transfer[188])MOV(8,Port_Data.Data_Transfer[189])SUB(K50.Command,9,SP_R_Index)OTL(Port_Data.Port_Read.[Port])OTL(Local_Control.4);
   37: XIO(Command_Being_Processed)XIO(Local_Control.4)EQU(K50.Command,14)[EQU(Type,2) ,EQU(Type,3) ]OTL(Command_Being_Processed)OTL(Local_Control.6);
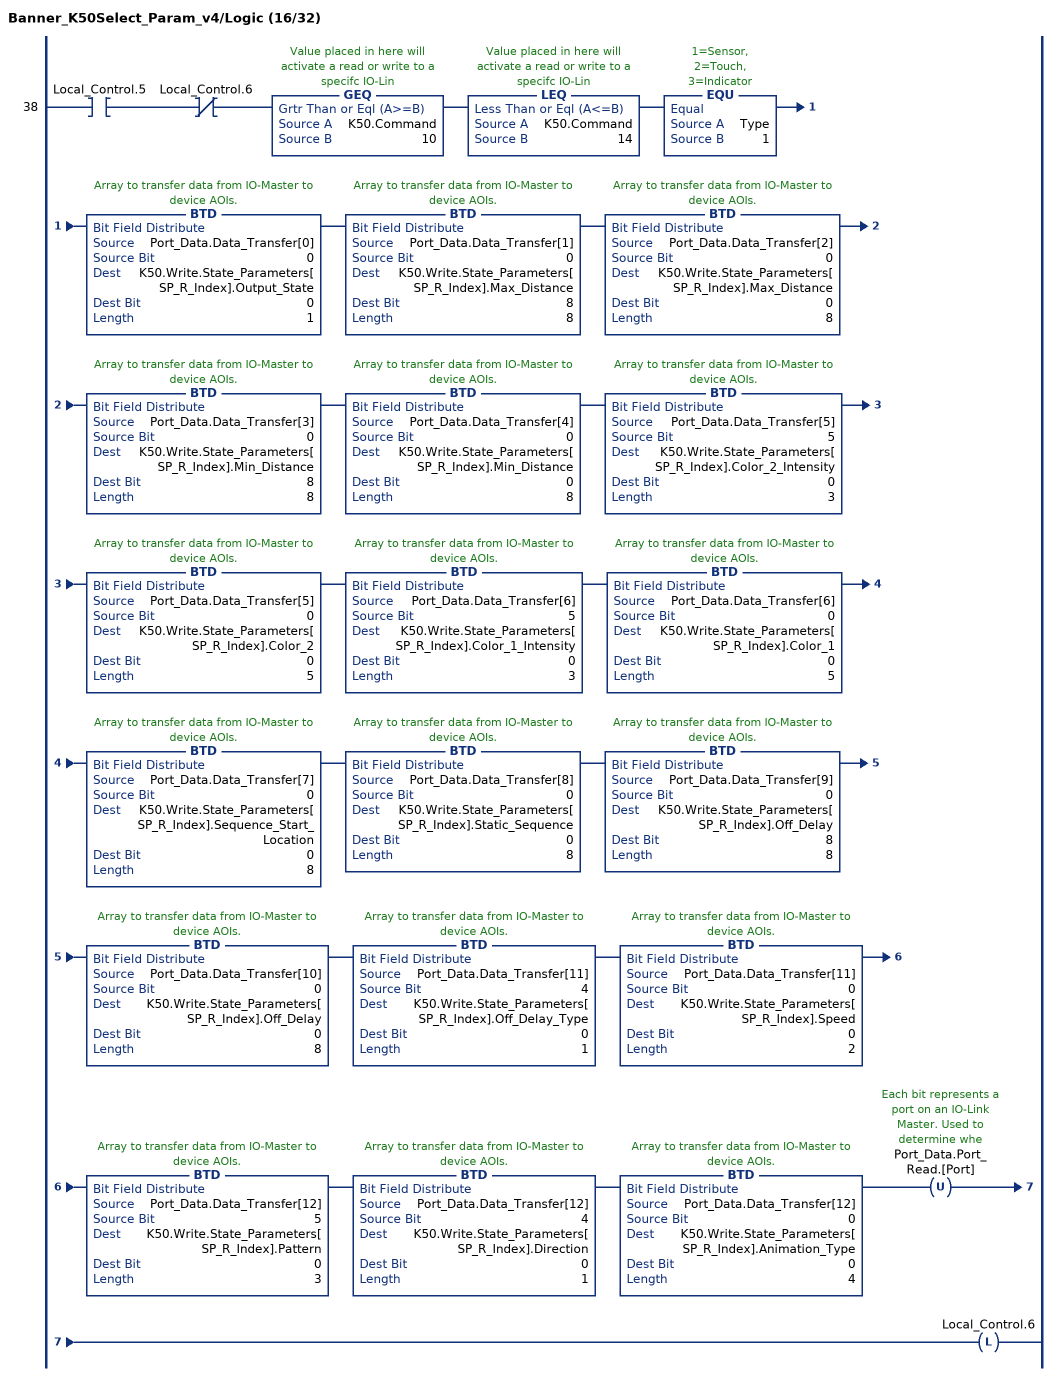
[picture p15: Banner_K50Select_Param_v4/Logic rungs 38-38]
   38: XIC(Local_Control.5)XIO(Local_Control.6)GEQ(K50.Command,10)LEQ(K50.Command,14)EQU(Type,1)BTD(Port_Data.Data_Transfer[0],0,K50.Write.State_Parameters[SP_R_Index].Output_State,0,1)BTD(Port_Data.Data_Transfer[1],0,K50.Write.State_Parameters[SP_R_Index].Max_Distance,8,8)BTD(Port_Data.Data_Transfer[2],0,K50.Write.State_Parameters[SP_R_Index].Max_Distance,0,8)BTD(Port_Data.Data_Transfer[3],0,K50.Write.State_Parameters[SP_R_Index].Min_Distance,8,8)BTD(Port_Data.Data_Transfer[4],0,K50.Write.State_Parameters[SP_R_Index].Min_Distance,0,8)BTD(Port_Data.Data_Transfer[5],5,K50.Write.State_Parameters[SP_R_Index].Color_2_Intensity,0,3)BTD(Port_Data.Data_Transfer[5],0,K50.Write.State_Parameters[SP_R_Index].Color_2,0,5)BTD(Port_Data.Data_Transfer[6],5,K50.Write.State_Parameters[SP_R_Index].Color_1_Intensity,0,3)BTD(Port_Data.Data_Transfer[6],0,K50.Write.State_Parameters[SP_R_Index].Color_1,0,5)BTD(Port_Data.Data_Transfer[7],0,K50.Write.State_Parameters[SP_R_Index].Sequence_Start_Location,0,8)BTD(Port_Data.Data_Transfer[8],0,K50.Write.State_Parameters[SP_R_Index].Static_Sequence,0,8)BTD(Port_Data.Data_Transfer[9],0,K50.Write.State_Parameters[SP_R_Index].Off_Delay,8,8)BTD(Port_Data.Data_Transfer[10],0,K50.Write.State_Parameters[SP_R_Index].Off_Delay,0,8)BTD(Port_Data.Data_Transfer[11],4,K50.Write.State_Parameters[SP_R_Index].Off_Delay_Type,0,1)BTD(Port_Data.Data_Transfer[11],0,K50.Write.State_Parameters[SP_R_Index].Speed,0,2)BTD(Port_Data.Data_Transfer[12],5,K50.Write.State_Parameters[SP_R_Index].Pattern,0,3)BTD(Port_Data.Data_Transfer[12],4,K50.Write.State_Parameters[SP_R_Index].Direction,0,1)BTD(Port_Data.Data_Transfer[12],0,K50.Write.State_Parameters[SP_R_Index].Animation_Type,0,4)OTU(Port_Data.Port_Read.[Port])OTL(Local_Control.6);
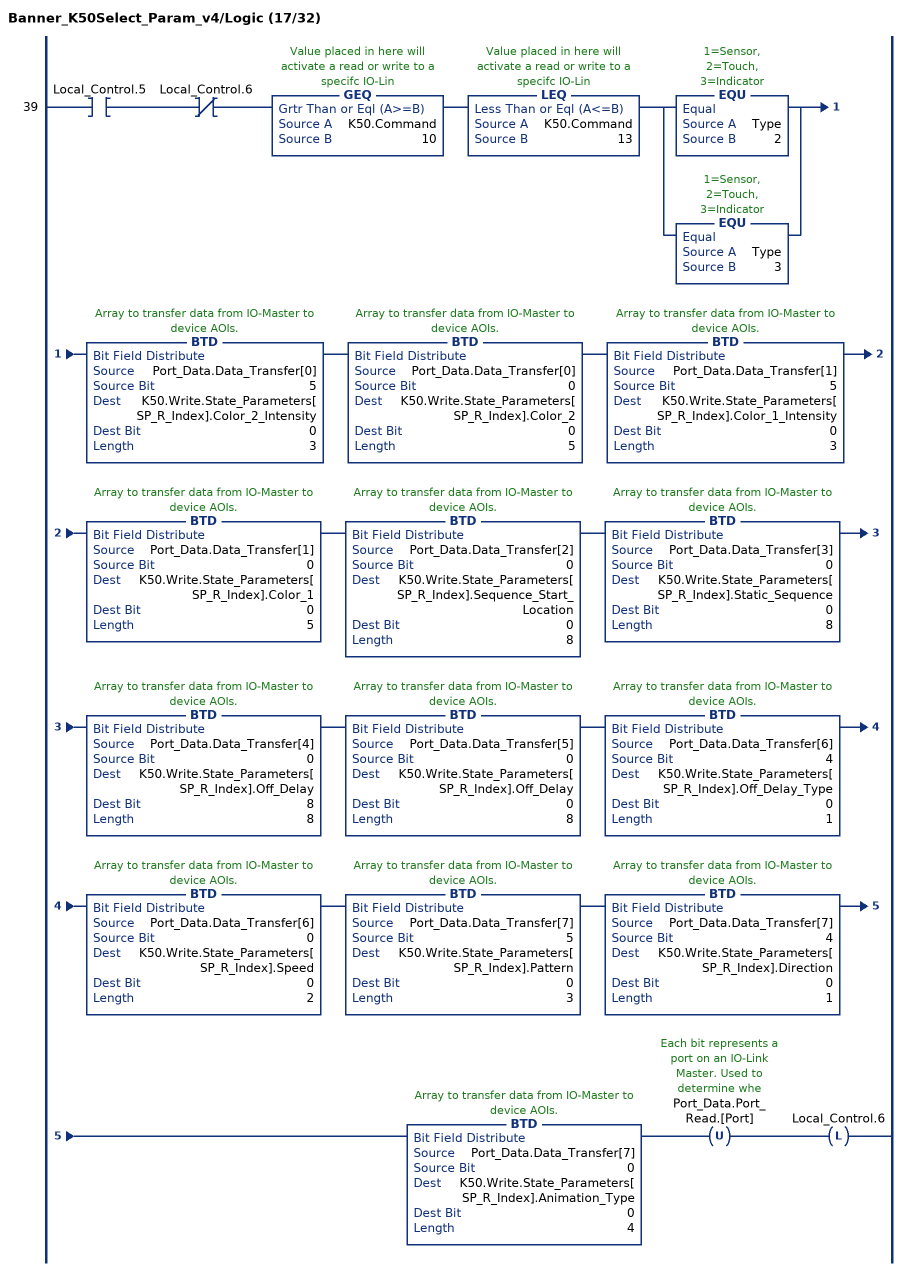
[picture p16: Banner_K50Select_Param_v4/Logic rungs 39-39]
   39: XIC(Local_Control.5)XIO(Local_Control.6)GEQ(K50.Command,10)LEQ(K50.Command,13)[EQU(Type,2) ,EQU(Type,3) ]BTD(Port_Data.Data_Transfer[0],5,K50.Write.State_Parameters[SP_R_Index].Color_2_Intensity,0,3)BTD(Port_Data.Data_Transfer[0],0,K50.Write.State_Parameters[SP_R_Index].Color_2,0,5)BTD(Port_Data.Data_Transfer[1],5,K50.Write.State_Parameters[SP_R_Index].Color_1_Intensity,0,3)BTD(Port_Data.Data_Transfer[1],0,K50.Write.State_Parameters[SP_R_Index].Color_1,0,5)BTD(Port_Data.Data_Transfer[2],0,K50.Write.State_Parameters[SP_R_Index].Sequence_Start_Location,0,8)BTD(Port_Data.Data_Transfer[3],0,K50.Write.State_Parameters[SP_R_Index].Static_Sequence,0,8)BTD(Port_Data.Data_Transfer[4],0,K50.Write.State_Parameters[SP_R_Index].Off_Delay,8,8)BTD(Port_Data.Data_Transfer[5],0,K50.Write.State_Parameters[SP_R_Index].Off_Delay,0,8)BTD(Port_Data.Data_Transfer[6],4,K50.Write.State_Parameters[SP_R_Index].Off_Delay_Type,0,1)BTD(Port_Data.Data_Transfer[6],0,K50.Write.State_Parameters[SP_R_Index].Speed,0,2)BTD(Port_Data.Data_Transfer[7],5,K50.Write.State_Parameters[SP_R_Index].Pattern,0,3)BTD(Port_Data.Data_Transfer[7],4,K50.Write.State_Parameters[SP_R_Index].Direction,0,1)BTD(Port_Data.Data_Transfer[7],0,K50.Write.State_Parameters[SP_R_Index].Animation_Type,0,4)OTU(Port_Data.Port_Read.[Port])OTL(Local_Control.6);
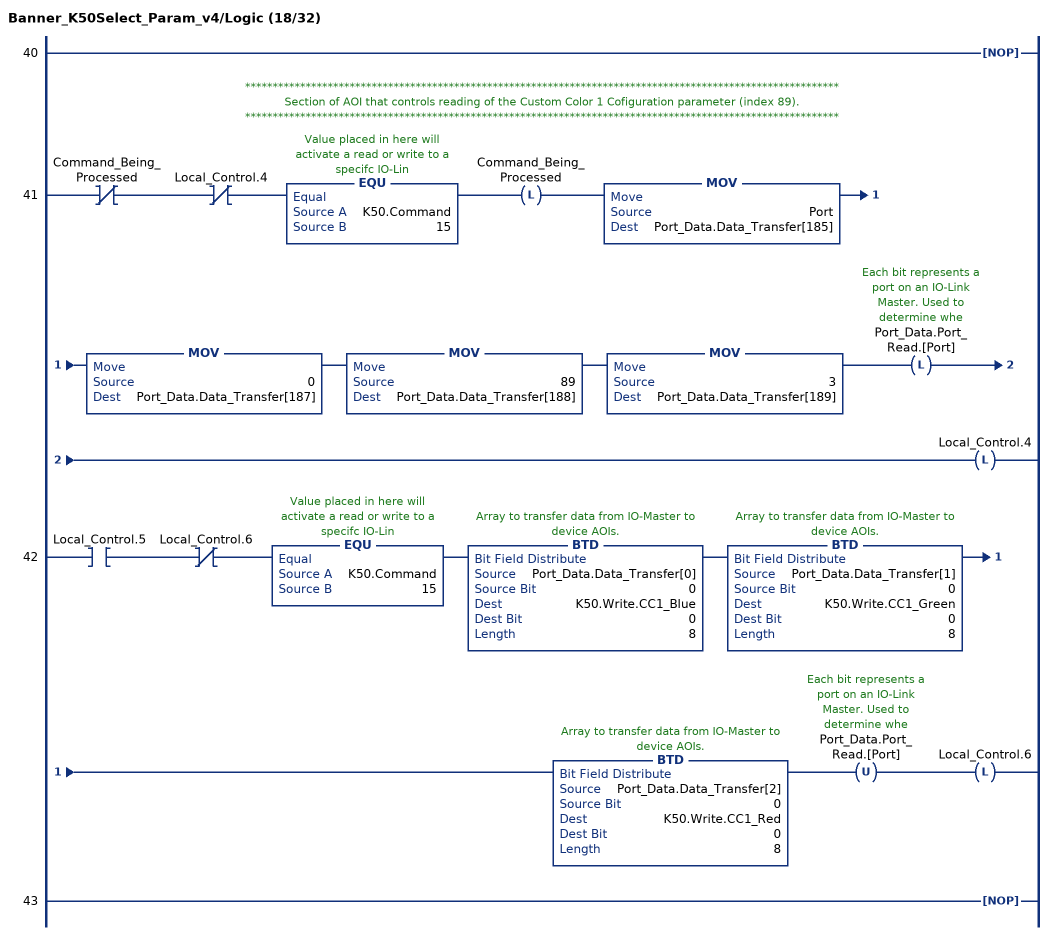
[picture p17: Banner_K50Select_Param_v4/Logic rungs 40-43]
   40: NOP();
   // ************************************************************************************************************
   // Section of AOI that controls reading of the Custom Color 1 Cofiguration parameter (index 89).
   // ************************************************************************************************************
   41: XIO(Command_Being_Processed)XIO(Local_Control.4)EQU(K50.Command,15)OTL(Command_Being_Processed)MOV(Port,Port_Data.Data_Transfer[185])MOV(0,Port_Data.Data_Transfer[187])MOV(89,Port_Data.Data_Transfer[188])MOV(3,Port_Data.Data_Transfer[189])OTL(Port_Data.Port_Read.[Port])OTL(Local_Control.4);
   42: XIC(Local_Control.5)XIO(Local_Control.6)EQU(K50.Command,15)BTD(Port_Data.Data_Transfer[0],0,K50.Write.CC1_Blue,0,8)BTD(Port_Data.Data_Transfer[1],0,K50.Write.CC1_Green,0,8)BTD(Port_Data.Data_Transfer[2],0,K50.Write.CC1_Red,0,8)OTU(Port_Data.Port_Read.[Port])OTL(Local_Control.6);
   43: NOP();
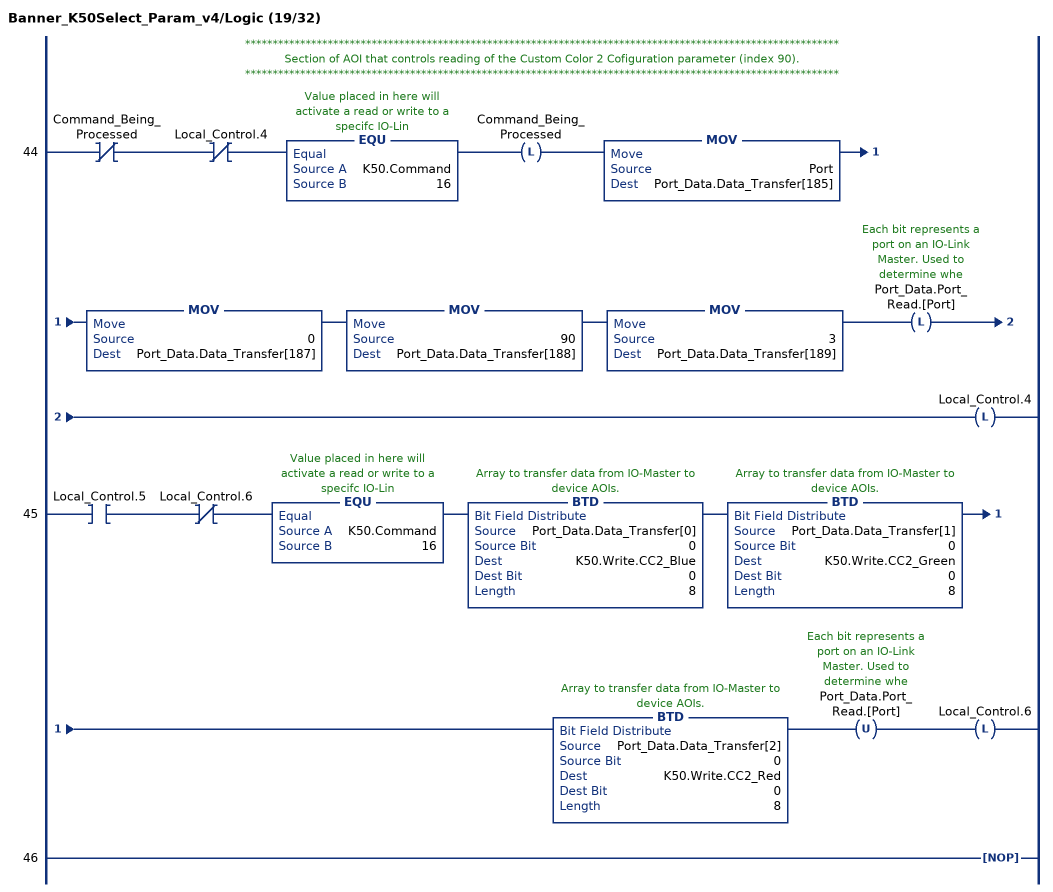
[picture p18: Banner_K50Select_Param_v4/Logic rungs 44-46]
   // ************************************************************************************************************
   // Section of AOI that controls reading of the Custom Color 2 Cofiguration parameter (index 90).
   // ************************************************************************************************************
   44: XIO(Command_Being_Processed)XIO(Local_Control.4)EQU(K50.Command,16)OTL(Command_Being_Processed)MOV(Port,Port_Data.Data_Transfer[185])MOV(0,Port_Data.Data_Transfer[187])MOV(90,Port_Data.Data_Transfer[188])MOV(3,Port_Data.Data_Transfer[189])OTL(Port_Data.Port_Read.[Port])OTL(Local_Control.4);
   45: XIC(Local_Control.5)XIO(Local_Control.6)EQU(K50.Command,16)BTD(Port_Data.Data_Transfer[0],0,K50.Write.CC2_Blue,0,8)BTD(Port_Data.Data_Transfer[1],0,K50.Write.CC2_Green,0,8)BTD(Port_Data.Data_Transfer[2],0,K50.Write.CC2_Red,0,8)OTU(Port_Data.Port_Read.[Port])OTL(Local_Control.6);
   46: NOP();
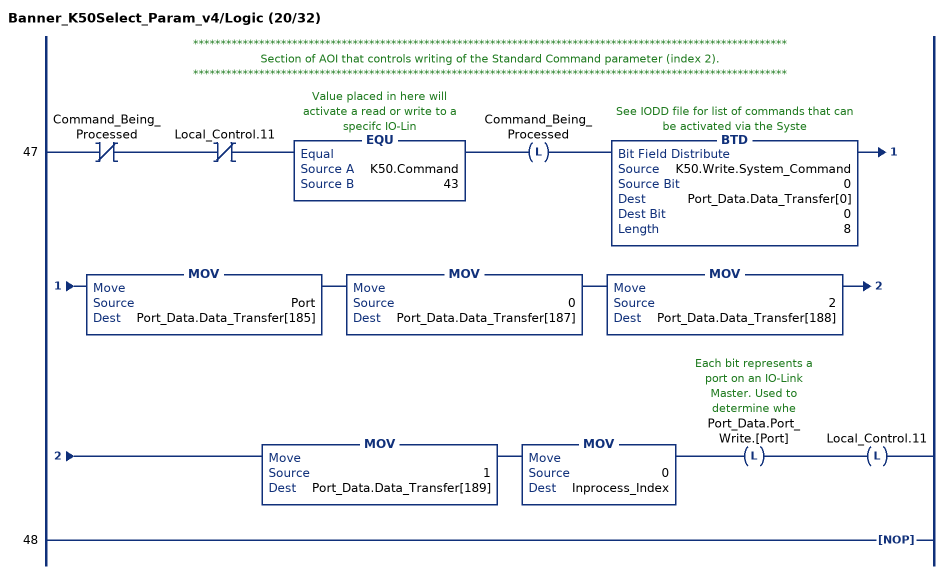
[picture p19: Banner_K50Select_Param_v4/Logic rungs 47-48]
   // ************************************************************************************************************
   // Section of AOI that controls writing of the Standard Command parameter (index 2).
   // ************************************************************************************************************
   47: XIO(Command_Being_Processed)XIO(Local_Control.11)EQU(K50.Command,43)OTL(Command_Being_Processed)BTD(K50.Write.System_Command,0,Port_Data.Data_Transfer[0],0,8)MOV(Port,Port_Data.Data_Transfer[185])MOV(0,Port_Data.Data_Transfer[187])MOV(2,Port_Data.Data_Transfer[188])MOV(1,Port_Data.Data_Transfer[189])MOV(0,Inprocess_Index)OTL(Port_Data.Port_Write.[Port])OTL(Local_Control.11);
   48: NOP();
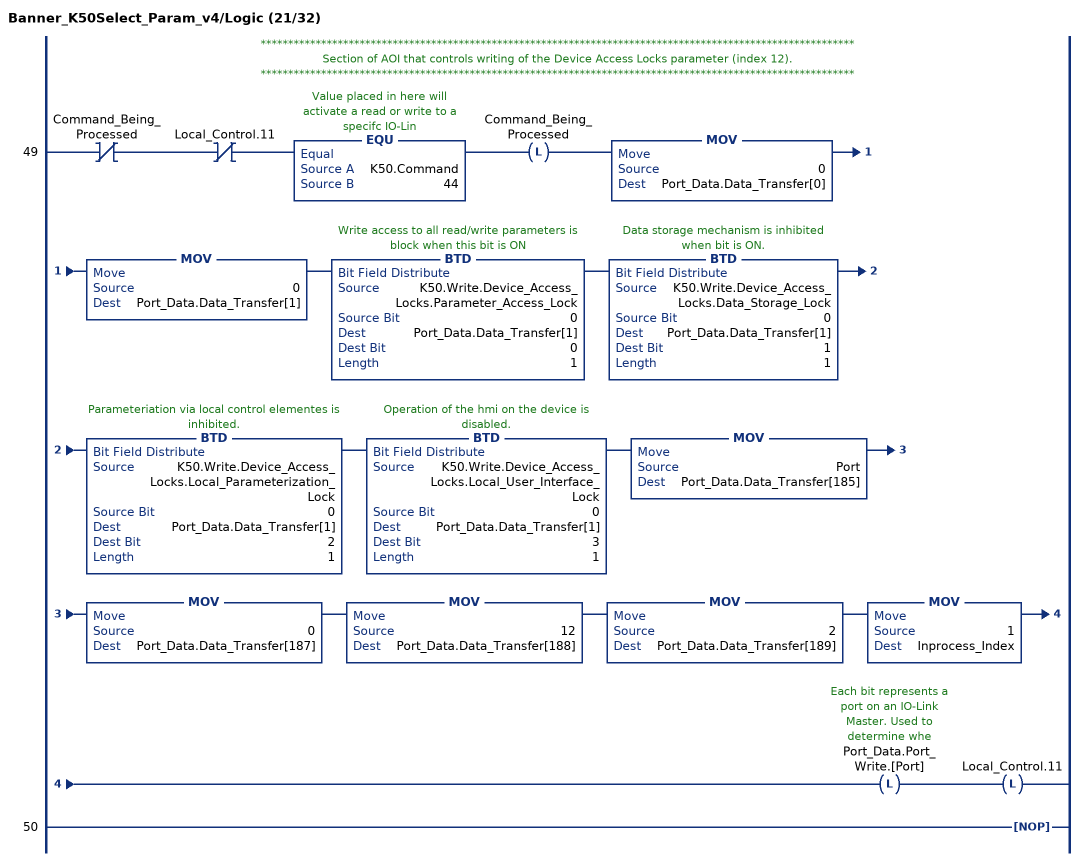
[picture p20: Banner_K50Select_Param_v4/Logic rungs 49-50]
   // ************************************************************************************************************
   // Section of AOI that controls writing of the Device Access Locks parameter (index 12).
   // ************************************************************************************************************
   49: XIO(Command_Being_Processed)XIO(Local_Control.11)EQU(K50.Command,44)OTL(Command_Being_Processed)MOV(0,Port_Data.Data_Transfer[0])MOV(0,Port_Data.Data_Transfer[1])BTD(K50.Write.Device_Access_Locks.Parameter_Access_Lock,0,Port_Data.Data_Transfer[1],0,1)BTD(K50.Write.Device_Access_Locks.Data_Storage_Lock,0,Port_Data.Data_Transfer[1],1,1)BTD(K50.Write.Device_Access_Locks.Local_Parameterization_Lock,0,Port_Data.Data_Transfer[1],2,1)BTD(K50.Write.Device_Access_Locks.Local_User_Interface_Lock,0,Port_Data.Data_Transfer[1],3,1)MOV(Port,Port_Data.Data_Transfer[185])MOV(0,Port_Data.Data_Transfer[187])MOV(12,Port_Data.Data_Transfer[188])MOV(2,Port_Data.Data_Transfer[189])MOV(1,Inprocess_Index)OTL(Port_Data.Port_Write.[Port])OTL(Local_Control.11);
   50: NOP();
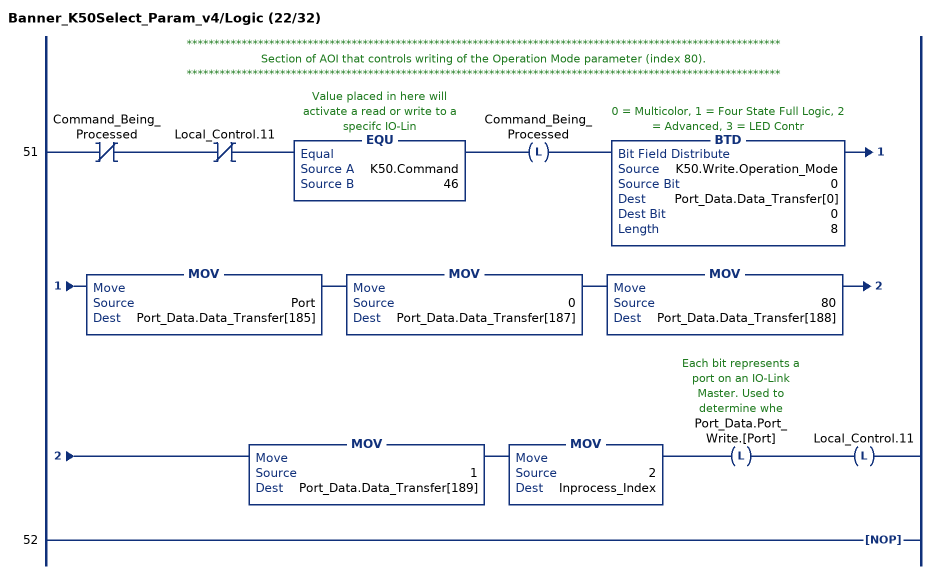
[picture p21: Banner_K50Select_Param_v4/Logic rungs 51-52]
   // ************************************************************************************************************
   // Section of AOI that controls writing of the Operation Mode parameter (index 80).
   // ************************************************************************************************************
   51: XIO(Command_Being_Processed)XIO(Local_Control.11)EQU(K50.Command,46)OTL(Command_Being_Processed)BTD(K50.Write.Operation_Mode,0,Port_Data.Data_Transfer[0],0,8)MOV(Port,Port_Data.Data_Transfer[185])MOV(0,Port_Data.Data_Transfer[187])MOV(80,Port_Data.Data_Transfer[188])MOV(1,Port_Data.Data_Transfer[189])MOV(2,Inprocess_Index)OTL(Port_Data.Port_Write.[Port])OTL(Local_Control.11);
   52: NOP();
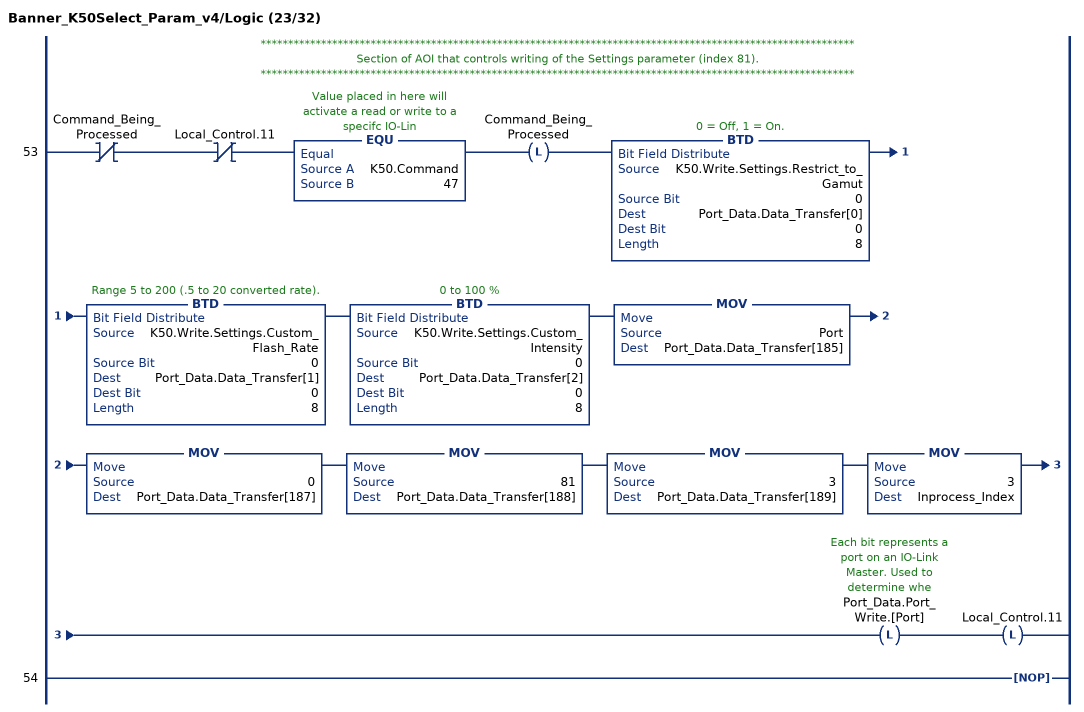
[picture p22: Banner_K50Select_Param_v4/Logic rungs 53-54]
   // ************************************************************************************************************
   // Section of AOI that controls writing of the Settings parameter (index 81).
   // ************************************************************************************************************
   53: XIO(Command_Being_Processed)XIO(Local_Control.11)EQU(K50.Command,47)OTL(Command_Being_Processed)BTD(K50.Write.Settings.Restrict_to_Gamut,0,Port_Data.Data_Transfer[0],0,8)BTD(K50.Write.Settings.Custom_Flash_Rate,0,Port_Data.Data_Transfer[1],0,8)BTD(K50.Write.Settings.Custom_Intensity,0,Port_Data.Data_Transfer[2],0,8)MOV(Port,Port_Data.Data_Transfer[185])MOV(0,Port_Data.Data_Transfer[187])MOV(81,Port_Data.Data_Transfer[188])MOV(3,Port_Data.Data_Transfer[189])MOV(3,Inprocess_Index)OTL(Port_Data.Port_Write.[Port])OTL(Local_Control.11);
   54: NOP();
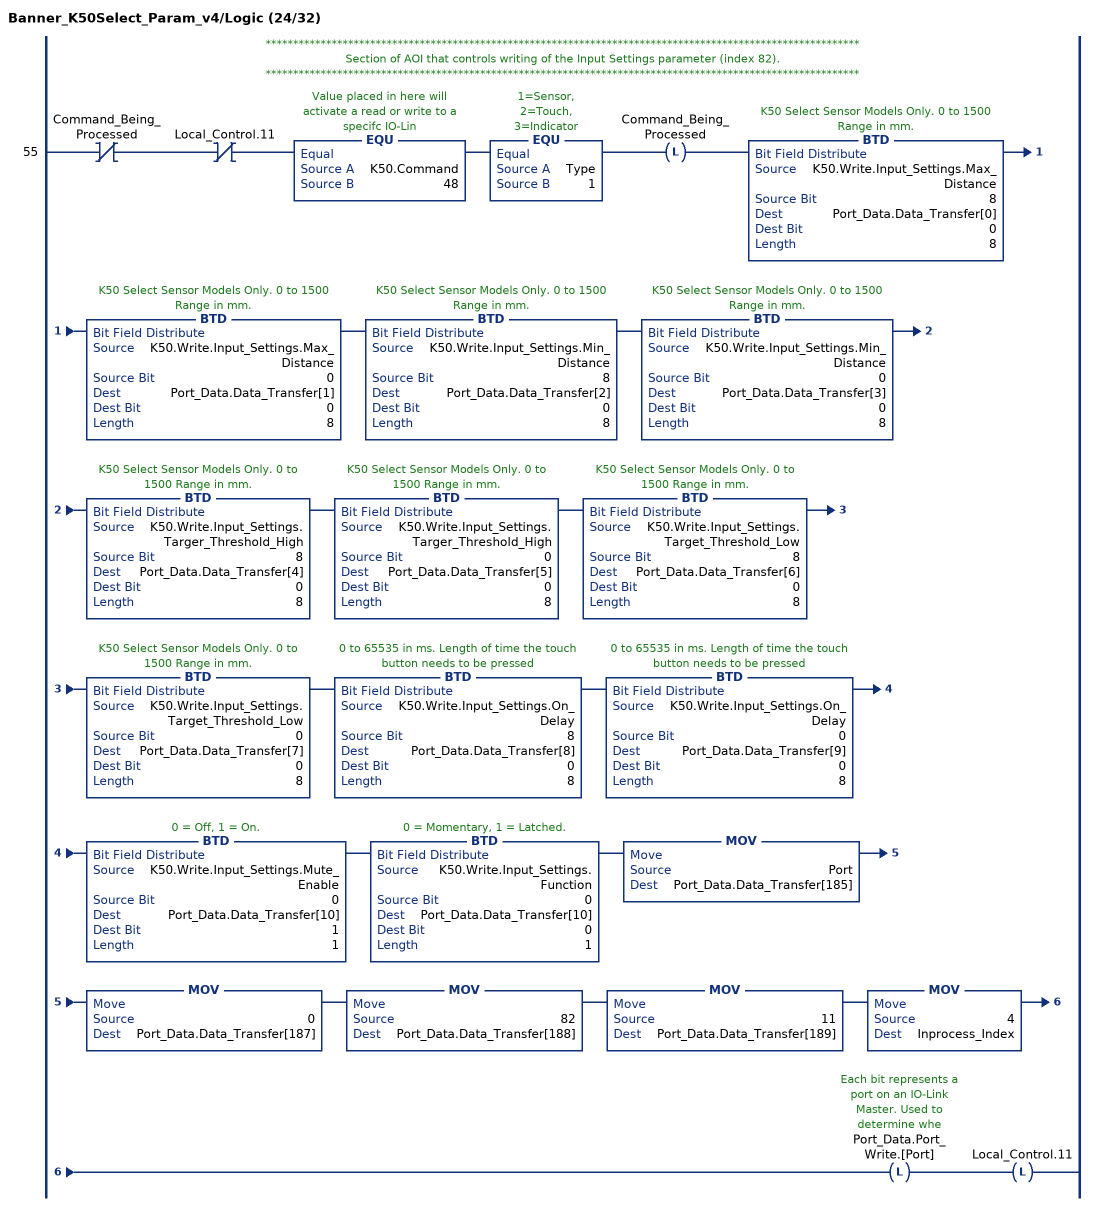
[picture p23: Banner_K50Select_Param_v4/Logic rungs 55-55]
   // ************************************************************************************************************
   // Section of AOI that controls writing of the Input Settings parameter (index 82).
   // ************************************************************************************************************
   55: XIO(Command_Being_Processed)XIO(Local_Control.11)EQU(K50.Command,48)EQU(Type,1)OTL(Command_Being_Processed)BTD(K50.Write.Input_Settings.Max_Distance,8,Port_Data.Data_Transfer[0],0,8)BTD(K50.Write.Input_Settings.Max_Distance,0,Port_Data.Data_Transfer[1],0,8)BTD(K50.Write.Input_Settings.Min_Distance,8,Port_Data.Data_Transfer[2],0,8)BTD(K50.Write.Input_Settings.Min_Distance,0,Port_Data.Data_Transfer[3],0,8)BTD(K50.Write.Input_Settings.Targer_Threshold_High,8,Port_Data.Data_Transfer[4],0,8)BTD(K50.Write.Input_Settings.Targer_Threshold_High,0,Port_Data.Data_Transfer[5],0,8)BTD(K50.Write.Input_Settings.Target_Threshold_Low,8,Port_Data.Data_Transfer[6],0,8)BTD(K50.Write.Input_Settings.Target_Threshold_Low,0,Port_Data.Data_Transfer[7],0,8)BTD(K50.Write.Input_Settings.On_Delay,8,Port_Data.Data_Transfer[8],0,8)BTD(K50.Write.Input_Settings.On_Delay,0,Port_Data.Data_Transfer[9],0,8)BTD(K50.Write.Input_Settings.Mute_Enable,0,Port_Data.Data_Transfer[10],1,1)BTD(K50.Write.Input_Settings.Function,0,Port_Data.Data_Transfer[10],0,1)MOV(Port,Port_Data.Data_Transfer[185])MOV(0,Port_Data.Data_Transfer[187])MOV(82,Port_Data.Data_Transfer[188])MOV(11,Port_Data.Data_Transfer[189])MOV(4,Inprocess_Index)OTL(Port_Data.Port_Write.[Port])OTL(Local_Control.11);
